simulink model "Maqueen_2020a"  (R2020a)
settings: Solver=VariableStepAuto  StartTime=0.0  StopTime=2  RelTol=1e-3
model workspace: external: MAT-File (data not in the file)
undefined symbols (not defined in the file or in its folder): deg, kg, m, mm, N, rad, s, smiData, X, Y, Z
libraries: sm_lib x459, fl_lib x12, nesl_utility x10
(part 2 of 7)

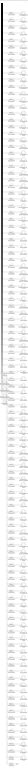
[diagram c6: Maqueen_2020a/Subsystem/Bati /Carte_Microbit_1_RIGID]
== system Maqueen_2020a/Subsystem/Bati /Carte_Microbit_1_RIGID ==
  Antenne_1_RIGID : Subsystem
  Assembly2_1_RIGID : Subsystem
  Button_assembly_microbit_1_RIGID : Subsystem
  Button_assembly_microbit_2_RIGID : Subsystem
  Button_assembly_microbit_3_RIGID : Subsystem
  Carte_microbit_1_RIGID : Subsystem
  Circuit_integre_1_1_RIGID : Subsystem
  Circuit_integre_2_1_RIGID : Subsystem
  Circuit_integre_3_1_RIGID : Subsystem
  Circuit_integre_3_2_RIGID : Subsystem
  Circuit_integre_4_1_RIGID : Subsystem
  Circuit_integre_4_2_RIGID : Subsystem
  Circuit_integre_5_1_RIGID : Subsystem
  Condensateur_1_RIGID : Subsystem
  Condensateur_2_RIGID : Subsystem
  Condensateur_3_RIGID : Subsystem
  Condensateur_4_RIGID : Subsystem
  Condensateur_5_RIGID : Subsystem
  Condensateur_6_RIGID : Subsystem
  Condensateur_cylindrique_10_RIGID : Subsystem
  Condensateur_cylindrique_11_RIGID : Subsystem
  Condensateur_cylindrique_12_RIGID : Subsystem
  Condensateur_cylindrique_13_RIGID : Subsystem
  Condensateur_cylindrique_14_RIGID : Subsystem
  Condensateur_cylindrique_15_RIGID : Subsystem
  Condensateur_cylindrique_16_RIGID : Subsystem
  Condensateur_cylindrique_17_RIGID : Subsystem
  Condensateur_cylindrique_18_RIGID : Subsystem
  Condensateur_cylindrique_19_RIGID : Subsystem
  Condensateur_cylindrique_1_RIGID : Subsystem
  Condensateur_cylindrique_20_RIGID : Subsystem
  Condensateur_cylindrique_2_RIGID : Subsystem
  Condensateur_cylindrique_3_RIGID : Subsystem
  Condensateur_cylindrique_4_RIGID : Subsystem
  Condensateur_cylindrique_5_RIGID : Subsystem
  Condensateur_cylindrique_6_RIGID : Subsystem
  Condensateur_cylindrique_7_RIGID : Subsystem
  Condensateur_cylindrique_8_RIGID : Subsystem
  Condensateur_cylindrique_9_RIGID : Subsystem
  Connecteur_alimentation_1_RIGID : Subsystem
  LED_10_RIGID : Subsystem
  LED_11_RIGID : Subsystem
  LED_12_RIGID : Subsystem
  LED_13_RIGID : Subsystem
  LED_14_RIGID : Subsystem
  LED_15_RIGID : Subsystem
  LED_16_RIGID : Subsystem
  LED_17_RIGID : Subsystem
  LED_18_RIGID : Subsystem
  LED_19_RIGID : Subsystem
  LED_1_RIGID : Subsystem
  LED_20_RIGID : Subsystem
  LED_21_RIGID : Subsystem
  LED_22_RIGID : Subsystem
  LED_23_RIGID : Subsystem
  LED_24_RIGID : Subsystem
  LED_25_RIGID : Subsystem
  LED_2_RIGID : Subsystem
  LED_3_RIGID : Subsystem
  LED_4_RIGID : Subsystem
  LED_5_RIGID : Subsystem
  LED_6_RIGID : Subsystem
  LED_7_RIGID : Subsystem
  LED_8_RIGID : Subsystem
  LED_9_RIGID : Subsystem
  Lignes_face_arrire_1_RIGID : Subsystem
  Pins_1_RIGID : Subsystem
  Pins_2_RIGID : Subsystem
  ReferenceFrame : sm_lib/Frames and Transforms/Reference Frame
  Resistance_10_RIGID : Subsystem
  Resistance_11_RIGID : Subsystem
  Resistance_12_RIGID : Subsystem
  Resistance_13_RIGID : Subsystem
  Resistance_14_RIGID : Subsystem
  Resistance_15_RIGID : Subsystem
  Resistance_16_RIGID : Subsystem
  Resistance_17_RIGID : Subsystem
  Resistance_18_RIGID : Subsystem
  Resistance_19_RIGID : Subsystem
  Resistance_1_RIGID : Subsystem
  Resistance_20_RIGID : Subsystem
  Resistance_21_RIGID : Subsystem
  Resistance_22_RIGID : Subsystem
  Resistance_23_RIGID : Subsystem
  Resistance_24_RIGID : Subsystem
  Resistance_25_RIGID : Subsystem
  Resistance_26_RIGID : Subsystem
  Resistance_27_RIGID : Subsystem
  Resistance_28_RIGID : Subsystem
  Resistance_29_RIGID : Subsystem
  Resistance_2_RIGID : Subsystem
  Resistance_30_RIGID : Subsystem
  Resistance_31_RIGID : Subsystem
  Resistance_32_RIGID : Subsystem
  Resistance_33_RIGID : Subsystem
  Resistance_34_RIGID : Subsystem
  Resistance_35_RIGID : Subsystem
  Resistance_36_RIGID : Subsystem
  Resistance_37_RIGID : Subsystem
  Resistance_38_RIGID : Subsystem
  Resistance_39_RIGID : Subsystem
  Resistance_3_RIGID : Subsystem
  Resistance_40_RIGID : Subsystem
  Resistance_41_RIGID : Subsystem
  Resistance_42_RIGID : Subsystem
  Resistance_43_RIGID : Subsystem
  Resistance_44_RIGID : Subsystem
  Resistance_45_RIGID : Subsystem
  Resistance_4_RIGID : Subsystem
  Resistance_5_RIGID : Subsystem
  Resistance_6_RIGID : Subsystem
  Resistance_7_RIGID : Subsystem
  Resistance_8_RIGID : Subsystem
  Resistance_9_RIGID : Subsystem
  Slot_condensateur_1_RIGID : Subsystem
  Texte_derriere_1_RIGID : Subsystem
  Texte_face_devant_1_RIGID : Subsystem
  Transform : sm_lib/Frames and Transforms/Rigid Transform  TranslationMethod=Cartesian  TranslationStandardOffset=0  TranslationLengthUnit=mm  TranslationStandardAxis=+Z  TranslationCartesianOffset=smiData.RigidTransform(6).translation  TranslationROffset=0  TranslationROffsetUnits=m  TranslationZOffset=0  TranslationZOffsetUnits=m  TranslationThetaOffset=0  TranslationThetaOffsetUnits=deg  RotationMethod=ArbitraryAxis  RotationAngleUnits=rad  RotationStandardAxis=+Z  RotationAngle=smiData.RigidTransform(6).angle  RotationArbitraryAxis=smiData.RigidTransform(6).axis  FollAlignAxisA=+X  BaseAlignAxisA=+Y  FollAlignAxisB=+Y  BaseAlignAxisB=+Z  RotationSequenceAxes=FollowerAxes  RotationSequence=XYX  RotationSequenceAngles=[0 0 0]  RotationSequenceAnglesUnits=deg  RotationMatrix=[1 0 0; 0 1 0; 0 0 1]
  Transform1 : sm_lib/Frames and Transforms/Rigid Transform  TranslationMethod=Cartesian  TranslationStandardOffset=0  TranslationLengthUnit=mm  TranslationStandardAxis=+Z  TranslationCartesianOffset=smiData.RigidTransform(29).translation  TranslationROffset=0  TranslationROffsetUnits=m  TranslationZOffset=0  TranslationZOffsetUnits=m  TranslationThetaOffset=0  TranslationThetaOffsetUnits=deg  RotationMethod=ArbitraryAxis  RotationAngleUnits=rad  RotationStandardAxis=+Z  RotationAngle=smiData.RigidTransform(29).angle  RotationArbitraryAxis=smiData.RigidTransform(29).axis  FollAlignAxisA=+X  BaseAlignAxisA=+Y  FollAlignAxisB=+Y  BaseAlignAxisB=+Z  RotationSequenceAxes=FollowerAxes  RotationSequence=XYX  RotationSequenceAngles=[0 0 0]  RotationSequenceAnglesUnits=deg  RotationMatrix=[1 0 0; 0 1 0; 0 0 1]
  Transform10 : sm_lib/Frames and Transforms/Rigid Transform  TranslationMethod=Cartesian  TranslationStandardOffset=0  TranslationLengthUnit=mm  TranslationStandardAxis=+Z  TranslationCartesianOffset=smiData.RigidTransform(38).translation  TranslationROffset=0  TranslationROffsetUnits=m  TranslationZOffset=0  TranslationZOffsetUnits=m  TranslationThetaOffset=0  TranslationThetaOffsetUnits=deg  RotationMethod=ArbitraryAxis  RotationAngleUnits=rad  RotationStandardAxis=+Z  RotationAngle=smiData.RigidTransform(38).angle  RotationArbitraryAxis=smiData.RigidTransform(38).axis  FollAlignAxisA=+X  BaseAlignAxisA=+Y  FollAlignAxisB=+Y  BaseAlignAxisB=+Z  RotationSequenceAxes=FollowerAxes  RotationSequence=XYX  RotationSequenceAngles=[0 0 0]  RotationSequenceAnglesUnits=deg  RotationMatrix=[1 0 0; 0 1 0; 0 0 1]
  Transform100 : sm_lib/Frames and Transforms/Rigid Transform  TranslationMethod=Cartesian  TranslationStandardOffset=0  TranslationLengthUnit=mm  TranslationStandardAxis=+Z  TranslationCartesianOffset=smiData.RigidTransform(137).translation  TranslationROffset=0  TranslationROffsetUnits=m  TranslationZOffset=0  TranslationZOffsetUnits=m  TranslationThetaOffset=0  TranslationThetaOffsetUnits=deg  RotationMethod=ArbitraryAxis  RotationAngleUnits=rad  RotationStandardAxis=+Z  RotationAngle=smiData.RigidTransform(137).angle  RotationArbitraryAxis=smiData.RigidTransform(137).axis  FollAlignAxisA=+X  BaseAlignAxisA=+Y  FollAlignAxisB=+Y  BaseAlignAxisB=+Z  RotationSequenceAxes=FollowerAxes  RotationSequence=XYX  RotationSequenceAngles=[0 0 0]  RotationSequenceAnglesUnits=deg  RotationMatrix=[1 0 0; 0 1 0; 0 0 1]
  Transform101 : sm_lib/Frames and Transforms/Rigid Transform  TranslationMethod=Cartesian  TranslationStandardOffset=0  TranslationLengthUnit=mm  TranslationStandardAxis=+Z  TranslationCartesianOffset=smiData.RigidTransform(138).translation  TranslationROffset=0  TranslationROffsetUnits=m  TranslationZOffset=0  TranslationZOffsetUnits=m  TranslationThetaOffset=0  TranslationThetaOffsetUnits=deg  RotationMethod=ArbitraryAxis  RotationAngleUnits=rad  RotationStandardAxis=+Z  RotationAngle=smiData.RigidTransform(138).angle  RotationArbitraryAxis=smiData.RigidTransform(138).axis  FollAlignAxisA=+X  BaseAlignAxisA=+Y  FollAlignAxisB=+Y  BaseAlignAxisB=+Z  RotationSequenceAxes=FollowerAxes  RotationSequence=XYX  RotationSequenceAngles=[0 0 0]  RotationSequenceAnglesUnits=deg  RotationMatrix=[1 0 0; 0 1 0; 0 0 1]
  Transform102 : sm_lib/Frames and Transforms/Rigid Transform  TranslationMethod=Cartesian  TranslationStandardOffset=0  TranslationLengthUnit=mm  TranslationStandardAxis=+Z  TranslationCartesianOffset=smiData.RigidTransform(139).translation  TranslationROffset=0  TranslationROffsetUnits=m  TranslationZOffset=0  TranslationZOffsetUnits=m  TranslationThetaOffset=0  TranslationThetaOffsetUnits=deg  RotationMethod=ArbitraryAxis  RotationAngleUnits=rad  RotationStandardAxis=+Z  RotationAngle=smiData.RigidTransform(139).angle  RotationArbitraryAxis=smiData.RigidTransform(139).axis  FollAlignAxisA=+X  BaseAlignAxisA=+Y  FollAlignAxisB=+Y  BaseAlignAxisB=+Z  RotationSequenceAxes=FollowerAxes  RotationSequence=XYX  RotationSequenceAngles=[0 0 0]  RotationSequenceAnglesUnits=deg  RotationMatrix=[1 0 0; 0 1 0; 0 0 1]
  Transform103 : sm_lib/Frames and Transforms/Rigid Transform  TranslationMethod=Cartesian  TranslationStandardOffset=0  TranslationLengthUnit=mm  TranslationStandardAxis=+Z  TranslationCartesianOffset=smiData.RigidTransform(140).translation  TranslationROffset=0  TranslationROffsetUnits=m  TranslationZOffset=0  TranslationZOffsetUnits=m  TranslationThetaOffset=0  TranslationThetaOffsetUnits=deg  RotationMethod=ArbitraryAxis  RotationAngleUnits=rad  RotationStandardAxis=+Z  RotationAngle=smiData.RigidTransform(140).angle  RotationArbitraryAxis=smiData.RigidTransform(140).axis  FollAlignAxisA=+X  BaseAlignAxisA=+Y  FollAlignAxisB=+Y  BaseAlignAxisB=+Z  RotationSequenceAxes=FollowerAxes  RotationSequence=XYX  RotationSequenceAngles=[0 0 0]  RotationSequenceAnglesUnits=deg  RotationMatrix=[1 0 0; 0 1 0; 0 0 1]
  Transform104 : sm_lib/Frames and Transforms/Rigid Transform  TranslationMethod=Cartesian  TranslationStandardOffset=0  TranslationLengthUnit=mm  TranslationStandardAxis=+Z  TranslationCartesianOffset=smiData.RigidTransform(145).translation  TranslationROffset=0  TranslationROffsetUnits=m  TranslationZOffset=0  TranslationZOffsetUnits=m  TranslationThetaOffset=0  TranslationThetaOffsetUnits=deg  RotationMethod=ArbitraryAxis  RotationAngleUnits=rad  RotationStandardAxis=+Z  RotationAngle=smiData.RigidTransform(145).angle  RotationArbitraryAxis=smiData.RigidTransform(145).axis  FollAlignAxisA=+X  BaseAlignAxisA=+Y  FollAlignAxisB=+Y  BaseAlignAxisB=+Z  RotationSequenceAxes=FollowerAxes  RotationSequence=XYX  RotationSequenceAngles=[0 0 0]  RotationSequenceAnglesUnits=deg  RotationMatrix=[1 0 0; 0 1 0; 0 0 1]
  Transform105 : sm_lib/Frames and Transforms/Rigid Transform  TranslationMethod=Cartesian  TranslationStandardOffset=0  TranslationLengthUnit=mm  TranslationStandardAxis=+Z  TranslationCartesianOffset=smiData.RigidTransform(150).translation  TranslationROffset=0  TranslationROffsetUnits=m  TranslationZOffset=0  TranslationZOffsetUnits=m  TranslationThetaOffset=0  TranslationThetaOffsetUnits=deg  RotationMethod=ArbitraryAxis  RotationAngleUnits=rad  RotationStandardAxis=+Z  RotationAngle=smiData.RigidTransform(150).angle  RotationArbitraryAxis=smiData.RigidTransform(150).axis  FollAlignAxisA=+X  BaseAlignAxisA=+Y  FollAlignAxisB=+Y  BaseAlignAxisB=+Z  RotationSequenceAxes=FollowerAxes  RotationSequence=XYX  RotationSequenceAngles=[0 0 0]  RotationSequenceAnglesUnits=deg  RotationMatrix=[1 0 0; 0 1 0; 0 0 1]
  Transform106 : sm_lib/Frames and Transforms/Rigid Transform  TranslationMethod=Cartesian  TranslationStandardOffset=0  TranslationLengthUnit=mm  TranslationStandardAxis=+Z  TranslationCartesianOffset=smiData.RigidTransform(151).translation  TranslationROffset=0  TranslationROffsetUnits=m  TranslationZOffset=0  TranslationZOffsetUnits=m  TranslationThetaOffset=0  TranslationThetaOffsetUnits=deg  RotationMethod=ArbitraryAxis  RotationAngleUnits=rad  RotationStandardAxis=+Z  RotationAngle=smiData.RigidTransform(151).angle  RotationArbitraryAxis=smiData.RigidTransform(151).axis  FollAlignAxisA=+X  BaseAlignAxisA=+Y  FollAlignAxisB=+Y  BaseAlignAxisB=+Z  RotationSequenceAxes=FollowerAxes  RotationSequence=XYX  RotationSequenceAngles=[0 0 0]  RotationSequenceAnglesUnits=deg  RotationMatrix=[1 0 0; 0 1 0; 0 0 1]
  Transform107 : sm_lib/Frames and Transforms/Rigid Transform  TranslationMethod=Cartesian  TranslationStandardOffset=0  TranslationLengthUnit=mm  TranslationStandardAxis=+Z  TranslationCartesianOffset=smiData.RigidTransform(152).translation  TranslationROffset=0  TranslationROffsetUnits=m  TranslationZOffset=0  TranslationZOffsetUnits=m  TranslationThetaOffset=0  TranslationThetaOffsetUnits=deg  RotationMethod=ArbitraryAxis  RotationAngleUnits=rad  RotationStandardAxis=+Z  RotationAngle=smiData.RigidTransform(152).angle  RotationArbitraryAxis=smiData.RigidTransform(152).axis  FollAlignAxisA=+X  BaseAlignAxisA=+Y  FollAlignAxisB=+Y  BaseAlignAxisB=+Z  RotationSequenceAxes=FollowerAxes  RotationSequence=XYX  RotationSequenceAngles=[0 0 0]  RotationSequenceAnglesUnits=deg  RotationMatrix=[1 0 0; 0 1 0; 0 0 1]
  Transform108 : sm_lib/Frames and Transforms/Rigid Transform  TranslationMethod=Cartesian  TranslationStandardOffset=0  TranslationLengthUnit=mm  TranslationStandardAxis=+Z  TranslationCartesianOffset=smiData.RigidTransform(153).translation  TranslationROffset=0  TranslationROffsetUnits=m  TranslationZOffset=0  TranslationZOffsetUnits=m  TranslationThetaOffset=0  TranslationThetaOffsetUnits=deg  RotationMethod=ArbitraryAxis  RotationAngleUnits=rad  RotationStandardAxis=+Z  RotationAngle=smiData.RigidTransform(153).angle  RotationArbitraryAxis=smiData.RigidTransform(153).axis  FollAlignAxisA=+X  BaseAlignAxisA=+Y  FollAlignAxisB=+Y  BaseAlignAxisB=+Z  RotationSequenceAxes=FollowerAxes  RotationSequence=XYX  RotationSequenceAngles=[0 0 0]  RotationSequenceAnglesUnits=deg  RotationMatrix=[1 0 0; 0 1 0; 0 0 1]
  Transform109 : sm_lib/Frames and Transforms/Rigid Transform  TranslationMethod=Cartesian  TranslationStandardOffset=0  TranslationLengthUnit=mm  TranslationStandardAxis=+Z  TranslationCartesianOffset=smiData.RigidTransform(154).translation  TranslationROffset=0  TranslationROffsetUnits=m  TranslationZOffset=0  TranslationZOffsetUnits=m  TranslationThetaOffset=0  TranslationThetaOffsetUnits=deg  RotationMethod=ArbitraryAxis  RotationAngleUnits=rad  RotationStandardAxis=+Z  RotationAngle=smiData.RigidTransform(154).angle  RotationArbitraryAxis=smiData.RigidTransform(154).axis  FollAlignAxisA=+X  BaseAlignAxisA=+Y  FollAlignAxisB=+Y  BaseAlignAxisB=+Z  RotationSequenceAxes=FollowerAxes  RotationSequence=XYX  RotationSequenceAngles=[0 0 0]  RotationSequenceAnglesUnits=deg  RotationMatrix=[1 0 0; 0 1 0; 0 0 1]
  Transform11 : sm_lib/Frames and Transforms/Rigid Transform  TranslationMethod=Cartesian  TranslationStandardOffset=0  TranslationLengthUnit=mm  TranslationStandardAxis=+Z  TranslationCartesianOffset=smiData.RigidTransform(39).translation  TranslationROffset=0  TranslationROffsetUnits=m  TranslationZOffset=0  TranslationZOffsetUnits=m  TranslationThetaOffset=0  TranslationThetaOffsetUnits=deg  RotationMethod=ArbitraryAxis  RotationAngleUnits=rad  RotationStandardAxis=+Z  RotationAngle=smiData.RigidTransform(39).angle  RotationArbitraryAxis=smiData.RigidTransform(39).axis  FollAlignAxisA=+X  BaseAlignAxisA=+Y  FollAlignAxisB=+Y  BaseAlignAxisB=+Z  RotationSequenceAxes=FollowerAxes  RotationSequence=XYX  RotationSequenceAngles=[0 0 0]  RotationSequenceAnglesUnits=deg  RotationMatrix=[1 0 0; 0 1 0; 0 0 1]
  Transform110 : sm_lib/Frames and Transforms/Rigid Transform  TranslationMethod=Cartesian  TranslationStandardOffset=0  TranslationLengthUnit=mm  TranslationStandardAxis=+Z  TranslationCartesianOffset=smiData.RigidTransform(155).translation  TranslationROffset=0  TranslationROffsetUnits=m  TranslationZOffset=0  TranslationZOffsetUnits=m  TranslationThetaOffset=0  TranslationThetaOffsetUnits=deg  RotationMethod=ArbitraryAxis  RotationAngleUnits=rad  RotationStandardAxis=+Z  RotationAngle=smiData.RigidTransform(155).angle  RotationArbitraryAxis=smiData.RigidTransform(155).axis  FollAlignAxisA=+X  BaseAlignAxisA=+Y  FollAlignAxisB=+Y  BaseAlignAxisB=+Z  RotationSequenceAxes=FollowerAxes  RotationSequence=XYX  RotationSequenceAngles=[0 0 0]  RotationSequenceAnglesUnits=deg  RotationMatrix=[1 0 0; 0 1 0; 0 0 1]
  Transform111 : sm_lib/Frames and Transforms/Rigid Transform  TranslationMethod=Cartesian  TranslationStandardOffset=0  TranslationLengthUnit=mm  TranslationStandardAxis=+Z  TranslationCartesianOffset=smiData.RigidTransform(156).translation  TranslationROffset=0  TranslationROffsetUnits=m  TranslationZOffset=0  TranslationZOffsetUnits=m  TranslationThetaOffset=0  TranslationThetaOffsetUnits=deg  RotationMethod=ArbitraryAxis  RotationAngleUnits=rad  RotationStandardAxis=+Z  RotationAngle=smiData.RigidTransform(156).angle  RotationArbitraryAxis=smiData.RigidTransform(156).axis  FollAlignAxisA=+X  BaseAlignAxisA=+Y  FollAlignAxisB=+Y  BaseAlignAxisB=+Z  RotationSequenceAxes=FollowerAxes  RotationSequence=XYX  RotationSequenceAngles=[0 0 0]  RotationSequenceAnglesUnits=deg  RotationMatrix=[1 0 0; 0 1 0; 0 0 1]
  Transform112 : sm_lib/Frames and Transforms/Rigid Transform  TranslationMethod=Cartesian  TranslationStandardOffset=0  TranslationLengthUnit=mm  TranslationStandardAxis=+Z  TranslationCartesianOffset=smiData.RigidTransform(157).translation  TranslationROffset=0  TranslationROffsetUnits=m  TranslationZOffset=0  TranslationZOffsetUnits=m  TranslationThetaOffset=0  TranslationThetaOffsetUnits=deg  RotationMethod=ArbitraryAxis  RotationAngleUnits=rad  RotationStandardAxis=+Z  RotationAngle=smiData.RigidTransform(157).angle  RotationArbitraryAxis=smiData.RigidTransform(157).axis  FollAlignAxisA=+X  BaseAlignAxisA=+Y  FollAlignAxisB=+Y  BaseAlignAxisB=+Z  RotationSequenceAxes=FollowerAxes  RotationSequence=XYX  RotationSequenceAngles=[0 0 0]  RotationSequenceAnglesUnits=deg  RotationMatrix=[1 0 0; 0 1 0; 0 0 1]
  Transform113 : sm_lib/Frames and Transforms/Rigid Transform  TranslationMethod=Cartesian  TranslationStandardOffset=0  TranslationLengthUnit=mm  TranslationStandardAxis=+Z  TranslationCartesianOffset=smiData.RigidTransform(158).translation  TranslationROffset=0  TranslationROffsetUnits=m  TranslationZOffset=0  TranslationZOffsetUnits=m  TranslationThetaOffset=0  TranslationThetaOffsetUnits=deg  RotationMethod=ArbitraryAxis  RotationAngleUnits=rad  RotationStandardAxis=+Z  RotationAngle=smiData.RigidTransform(158).angle  RotationArbitraryAxis=smiData.RigidTransform(158).axis  FollAlignAxisA=+X  BaseAlignAxisA=+Y  FollAlignAxisB=+Y  BaseAlignAxisB=+Z  RotationSequenceAxes=FollowerAxes  RotationSequence=XYX  RotationSequenceAngles=[0 0 0]  RotationSequenceAnglesUnits=deg  RotationMatrix=[1 0 0; 0 1 0; 0 0 1]
  Transform12 : sm_lib/Frames and Transforms/Rigid Transform  TranslationMethod=Cartesian  TranslationStandardOffset=0  TranslationLengthUnit=mm  TranslationStandardAxis=+Z  TranslationCartesianOffset=smiData.RigidTransform(40).translation  TranslationROffset=0  TranslationROffsetUnits=m  TranslationZOffset=0  TranslationZOffsetUnits=m  TranslationThetaOffset=0  TranslationThetaOffsetUnits=deg  RotationMethod=ArbitraryAxis  RotationAngleUnits=rad  RotationStandardAxis=+Z  RotationAngle=smiData.RigidTransform(40).angle  RotationArbitraryAxis=smiData.RigidTransform(40).axis  FollAlignAxisA=+X  BaseAlignAxisA=+Y  FollAlignAxisB=+Y  BaseAlignAxisB=+Z  RotationSequenceAxes=FollowerAxes  RotationSequence=XYX  RotationSequenceAngles=[0 0 0]  RotationSequenceAnglesUnits=deg  RotationMatrix=[1 0 0; 0 1 0; 0 0 1]
  Transform13 : sm_lib/Frames and Transforms/Rigid Transform  TranslationMethod=Cartesian  TranslationStandardOffset=0  TranslationLengthUnit=mm  TranslationStandardAxis=+Z  TranslationCartesianOffset=smiData.RigidTransform(41).translation  TranslationROffset=0  TranslationROffsetUnits=m  TranslationZOffset=0  TranslationZOffsetUnits=m  TranslationThetaOffset=0  TranslationThetaOffsetUnits=deg  RotationMethod=ArbitraryAxis  RotationAngleUnits=rad  RotationStandardAxis=+Z  RotationAngle=smiData.RigidTransform(41).angle  RotationArbitraryAxis=smiData.RigidTransform(41).axis  FollAlignAxisA=+X  BaseAlignAxisA=+Y  FollAlignAxisB=+Y  BaseAlignAxisB=+Z  RotationSequenceAxes=FollowerAxes  RotationSequence=XYX  RotationSequenceAngles=[0 0 0]  RotationSequenceAnglesUnits=deg  RotationMatrix=[1 0 0; 0 1 0; 0 0 1]
  Transform14 : sm_lib/Frames and Transforms/Rigid Transform  TranslationMethod=Cartesian  TranslationStandardOffset=0  TranslationLengthUnit=mm  TranslationStandardAxis=+Z  TranslationCartesianOffset=smiData.RigidTransform(42).translation  TranslationROffset=0  TranslationROffsetUnits=m  TranslationZOffset=0  TranslationZOffsetUnits=m  TranslationThetaOffset=0  TranslationThetaOffsetUnits=deg  RotationMethod=ArbitraryAxis  RotationAngleUnits=rad  RotationStandardAxis=+Z  RotationAngle=smiData.RigidTransform(42).angle  RotationArbitraryAxis=smiData.RigidTransform(42).axis  FollAlignAxisA=+X  BaseAlignAxisA=+Y  FollAlignAxisB=+Y  BaseAlignAxisB=+Z  RotationSequenceAxes=FollowerAxes  RotationSequence=XYX  RotationSequenceAngles=[0 0 0]  RotationSequenceAnglesUnits=deg  RotationMatrix=[1 0 0; 0 1 0; 0 0 1]
  Transform15 : sm_lib/Frames and Transforms/Rigid Transform  TranslationMethod=Cartesian  TranslationStandardOffset=0  TranslationLengthUnit=mm  TranslationStandardAxis=+Z  TranslationCartesianOffset=smiData.RigidTransform(43).translation  TranslationROffset=0  TranslationROffsetUnits=m  TranslationZOffset=0  TranslationZOffsetUnits=m  TranslationThetaOffset=0  TranslationThetaOffsetUnits=deg  RotationMethod=ArbitraryAxis  RotationAngleUnits=rad  RotationStandardAxis=+Z  RotationAngle=smiData.RigidTransform(43).angle  RotationArbitraryAxis=smiData.RigidTransform(43).axis  FollAlignAxisA=+X  BaseAlignAxisA=+Y  FollAlignAxisB=+Y  BaseAlignAxisB=+Z  RotationSequenceAxes=FollowerAxes  RotationSequence=XYX  RotationSequenceAngles=[0 0 0]  RotationSequenceAnglesUnits=deg  RotationMatrix=[1 0 0; 0 1 0; 0 0 1]
  Transform16 : sm_lib/Frames and Transforms/Rigid Transform  TranslationMethod=Cartesian  TranslationStandardOffset=0  TranslationLengthUnit=mm  TranslationStandardAxis=+Z  TranslationCartesianOffset=smiData.RigidTransform(44).translation  TranslationROffset=0  TranslationROffsetUnits=m  TranslationZOffset=0  TranslationZOffsetUnits=m  TranslationThetaOffset=0  TranslationThetaOffsetUnits=deg  RotationMethod=ArbitraryAxis  RotationAngleUnits=rad  RotationStandardAxis=+Z  RotationAngle=smiData.RigidTransform(44).angle  RotationArbitraryAxis=smiData.RigidTransform(44).axis  FollAlignAxisA=+X  BaseAlignAxisA=+Y  FollAlignAxisB=+Y  BaseAlignAxisB=+Z  RotationSequenceAxes=FollowerAxes  RotationSequence=XYX  RotationSequenceAngles=[0 0 0]  RotationSequenceAnglesUnits=deg  RotationMatrix=[1 0 0; 0 1 0; 0 0 1]
  Transform17 : sm_lib/Frames and Transforms/Rigid Transform  TranslationMethod=Cartesian  TranslationStandardOffset=0  TranslationLengthUnit=mm  TranslationStandardAxis=+Z  TranslationCartesianOffset=smiData.RigidTransform(45).translation  TranslationROffset=0  TranslationROffsetUnits=m  TranslationZOffset=0  TranslationZOffsetUnits=m  TranslationThetaOffset=0  TranslationThetaOffsetUnits=deg  RotationMethod=ArbitraryAxis  RotationAngleUnits=rad  RotationStandardAxis=+Z  RotationAngle=smiData.RigidTransform(45).angle  RotationArbitraryAxis=smiData.RigidTransform(45).axis  FollAlignAxisA=+X  BaseAlignAxisA=+Y  FollAlignAxisB=+Y  BaseAlignAxisB=+Z  RotationSequenceAxes=FollowerAxes  RotationSequence=XYX  RotationSequenceAngles=[0 0 0]  RotationSequenceAnglesUnits=deg  RotationMatrix=[1 0 0; 0 1 0; 0 0 1]
  Transform18 : sm_lib/Frames and Transforms/Rigid Transform  TranslationMethod=Cartesian  TranslationStandardOffset=0  TranslationLengthUnit=mm  TranslationStandardAxis=+Z  TranslationCartesianOffset=smiData.RigidTransform(46).translation  TranslationROffset=0  TranslationROffsetUnits=m  TranslationZOffset=0  TranslationZOffsetUnits=m  TranslationThetaOffset=0  TranslationThetaOffsetUnits=deg  RotationMethod=ArbitraryAxis  RotationAngleUnits=rad  RotationStandardAxis=+Z  RotationAngle=smiData.RigidTransform(46).angle  RotationArbitraryAxis=smiData.RigidTransform(46).axis  FollAlignAxisA=+X  BaseAlignAxisA=+Y  FollAlignAxisB=+Y  BaseAlignAxisB=+Z  RotationSequenceAxes=FollowerAxes  RotationSequence=XYX  RotationSequenceAngles=[0 0 0]  RotationSequenceAnglesUnits=deg  RotationMatrix=[1 0 0; 0 1 0; 0 0 1]
  Transform19 : sm_lib/Frames and Transforms/Rigid Transform  TranslationMethod=Cartesian  TranslationStandardOffset=0  TranslationLengthUnit=mm  TranslationStandardAxis=+Z  TranslationCartesianOffset=smiData.RigidTransform(47).translation  TranslationROffset=0  TranslationROffsetUnits=m  TranslationZOffset=0  TranslationZOffsetUnits=m  TranslationThetaOffset=0  TranslationThetaOffsetUnits=deg  RotationMethod=ArbitraryAxis  RotationAngleUnits=rad  RotationStandardAxis=+Z  RotationAngle=smiData.RigidTransform(47).angle  RotationArbitraryAxis=smiData.RigidTransform(47).axis  FollAlignAxisA=+X  BaseAlignAxisA=+Y  FollAlignAxisB=+Y  BaseAlignAxisB=+Z  RotationSequenceAxes=FollowerAxes  RotationSequence=XYX  RotationSequenceAngles=[0 0 0]  RotationSequenceAnglesUnits=deg  RotationMatrix=[1 0 0; 0 1 0; 0 0 1]
  Transform2 : sm_lib/Frames and Transforms/Rigid Transform  TranslationMethod=Cartesian  TranslationStandardOffset=0  TranslationLengthUnit=mm  TranslationStandardAxis=+Z  TranslationCartesianOffset=smiData.RigidTransform(30).translation  TranslationROffset=0  TranslationROffsetUnits=m  TranslationZOffset=0  TranslationZOffsetUnits=m  TranslationThetaOffset=0  TranslationThetaOffsetUnits=deg  RotationMethod=ArbitraryAxis  RotationAngleUnits=rad  RotationStandardAxis=+Z  RotationAngle=smiData.RigidTransform(30).angle  RotationArbitraryAxis=smiData.RigidTransform(30).axis  FollAlignAxisA=+X  BaseAlignAxisA=+Y  FollAlignAxisB=+Y  BaseAlignAxisB=+Z  RotationSequenceAxes=FollowerAxes  RotationSequence=XYX  RotationSequenceAngles=[0 0 0]  RotationSequenceAnglesUnits=deg  RotationMatrix=[1 0 0; 0 1 0; 0 0 1]
  Transform20 : sm_lib/Frames and Transforms/Rigid Transform  TranslationMethod=Cartesian  TranslationStandardOffset=0  TranslationLengthUnit=mm  TranslationStandardAxis=+Z  TranslationCartesianOffset=smiData.RigidTransform(48).translation  TranslationROffset=0  TranslationROffsetUnits=m  TranslationZOffset=0  TranslationZOffsetUnits=m  TranslationThetaOffset=0  TranslationThetaOffsetUnits=deg  RotationMethod=ArbitraryAxis  RotationAngleUnits=rad  RotationStandardAxis=+Z  RotationAngle=smiData.RigidTransform(48).angle  RotationArbitraryAxis=smiData.RigidTransform(48).axis  FollAlignAxisA=+X  BaseAlignAxisA=+Y  FollAlignAxisB=+Y  BaseAlignAxisB=+Z  RotationSequenceAxes=FollowerAxes  RotationSequence=XYX  RotationSequenceAngles=[0 0 0]  RotationSequenceAnglesUnits=deg  RotationMatrix=[1 0 0; 0 1 0; 0 0 1]
  Transform21 : sm_lib/Frames and Transforms/Rigid Transform  TranslationMethod=Cartesian  TranslationStandardOffset=0  TranslationLengthUnit=mm  TranslationStandardAxis=+Z  TranslationCartesianOffset=smiData.RigidTransform(49).translation  TranslationROffset=0  TranslationROffsetUnits=m  TranslationZOffset=0  TranslationZOffsetUnits=m  TranslationThetaOffset=0  TranslationThetaOffsetUnits=deg  RotationMethod=ArbitraryAxis  RotationAngleUnits=rad  RotationStandardAxis=+Z  RotationAngle=smiData.RigidTransform(49).angle  RotationArbitraryAxis=smiData.RigidTransform(49).axis  FollAlignAxisA=+X  BaseAlignAxisA=+Y  FollAlignAxisB=+Y  BaseAlignAxisB=+Z  RotationSequenceAxes=FollowerAxes  RotationSequence=XYX  RotationSequenceAngles=[0 0 0]  RotationSequenceAnglesUnits=deg  RotationMatrix=[1 0 0; 0 1 0; 0 0 1]
  Transform22 : sm_lib/Frames and Transforms/Rigid Transform  TranslationMethod=Cartesian  TranslationStandardOffset=0  TranslationLengthUnit=mm  TranslationStandardAxis=+Z  TranslationCartesianOffset=smiData.RigidTransform(50).translation  TranslationROffset=0  TranslationROffsetUnits=m  TranslationZOffset=0  TranslationZOffsetUnits=m  TranslationThetaOffset=0  TranslationThetaOffsetUnits=deg  RotationMethod=ArbitraryAxis  RotationAngleUnits=rad  RotationStandardAxis=+Z  RotationAngle=smiData.RigidTransform(50).angle  RotationArbitraryAxis=smiData.RigidTransform(50).axis  FollAlignAxisA=+X  BaseAlignAxisA=+Y  FollAlignAxisB=+Y  BaseAlignAxisB=+Z  RotationSequenceAxes=FollowerAxes  RotationSequence=XYX  RotationSequenceAngles=[0 0 0]  RotationSequenceAnglesUnits=deg  RotationMatrix=[1 0 0; 0 1 0; 0 0 1]
  Transform23 : sm_lib/Frames and Transforms/Rigid Transform  TranslationMethod=Cartesian  TranslationStandardOffset=0  TranslationLengthUnit=mm  TranslationStandardAxis=+Z  TranslationCartesianOffset=smiData.RigidTransform(51).translation  TranslationROffset=0  TranslationROffsetUnits=m  TranslationZOffset=0  TranslationZOffsetUnits=m  TranslationThetaOffset=0  TranslationThetaOffsetUnits=deg  RotationMethod=ArbitraryAxis  RotationAngleUnits=rad  RotationStandardAxis=+Z  RotationAngle=smiData.RigidTransform(51).angle  RotationArbitraryAxis=smiData.RigidTransform(51).axis  FollAlignAxisA=+X  BaseAlignAxisA=+Y  FollAlignAxisB=+Y  BaseAlignAxisB=+Z  RotationSequenceAxes=FollowerAxes  RotationSequence=XYX  RotationSequenceAngles=[0 0 0]  RotationSequenceAnglesUnits=deg  RotationMatrix=[1 0 0; 0 1 0; 0 0 1]
  Transform24 : sm_lib/Frames and Transforms/Rigid Transform  TranslationMethod=Cartesian  TranslationStandardOffset=0  TranslationLengthUnit=mm  TranslationStandardAxis=+Z  TranslationCartesianOffset=smiData.RigidTransform(52).translation  TranslationROffset=0  TranslationROffsetUnits=m  TranslationZOffset=0  TranslationZOffsetUnits=m  TranslationThetaOffset=0  TranslationThetaOffsetUnits=deg  RotationMethod=ArbitraryAxis  RotationAngleUnits=rad  RotationStandardAxis=+Z  RotationAngle=smiData.RigidTransform(52).angle  RotationArbitraryAxis=smiData.RigidTransform(52).axis  FollAlignAxisA=+X  BaseAlignAxisA=+Y  FollAlignAxisB=+Y  BaseAlignAxisB=+Z  RotationSequenceAxes=FollowerAxes  RotationSequence=XYX  RotationSequenceAngles=[0 0 0]  RotationSequenceAnglesUnits=deg  RotationMatrix=[1 0 0; 0 1 0; 0 0 1]
  Transform25 : sm_lib/Frames and Transforms/Rigid Transform  TranslationMethod=Cartesian  TranslationStandardOffset=0  TranslationLengthUnit=mm  TranslationStandardAxis=+Z  TranslationCartesianOffset=smiData.RigidTransform(53).translation  TranslationROffset=0  TranslationROffsetUnits=m  TranslationZOffset=0  TranslationZOffsetUnits=m  TranslationThetaOffset=0  TranslationThetaOffsetUnits=deg  RotationMethod=ArbitraryAxis  RotationAngleUnits=rad  RotationStandardAxis=+Z  RotationAngle=smiData.RigidTransform(53).angle  RotationArbitraryAxis=smiData.RigidTransform(53).axis  FollAlignAxisA=+X  BaseAlignAxisA=+Y  FollAlignAxisB=+Y  BaseAlignAxisB=+Z  RotationSequenceAxes=FollowerAxes  RotationSequence=XYX  RotationSequenceAngles=[0 0 0]  RotationSequenceAnglesUnits=deg  RotationMatrix=[1 0 0; 0 1 0; 0 0 1]
  Transform26 : sm_lib/Frames and Transforms/Rigid Transform  TranslationMethod=Cartesian  TranslationStandardOffset=0  TranslationLengthUnit=mm  TranslationStandardAxis=+Z  TranslationCartesianOffset=smiData.RigidTransform(54).translation  TranslationROffset=0  TranslationROffsetUnits=m  TranslationZOffset=0  TranslationZOffsetUnits=m  TranslationThetaOffset=0  TranslationThetaOffsetUnits=deg  RotationMethod=ArbitraryAxis  RotationAngleUnits=rad  RotationStandardAxis=+Z  RotationAngle=smiData.RigidTransform(54).angle  RotationArbitraryAxis=smiData.RigidTransform(54).axis  FollAlignAxisA=+X  BaseAlignAxisA=+Y  FollAlignAxisB=+Y  BaseAlignAxisB=+Z  RotationSequenceAxes=FollowerAxes  RotationSequence=XYX  RotationSequenceAngles=[0 0 0]  RotationSequenceAnglesUnits=deg  RotationMatrix=[1 0 0; 0 1 0; 0 0 1]
  Transform27 : sm_lib/Frames and Transforms/Rigid Transform  TranslationMethod=Cartesian  TranslationStandardOffset=0  TranslationLengthUnit=mm  TranslationStandardAxis=+Z  TranslationCartesianOffset=smiData.RigidTransform(55).translation  TranslationROffset=0  TranslationROffsetUnits=m  TranslationZOffset=0  TranslationZOffsetUnits=m  TranslationThetaOffset=0  TranslationThetaOffsetUnits=deg  RotationMethod=ArbitraryAxis  RotationAngleUnits=rad  RotationStandardAxis=+Z  RotationAngle=smiData.RigidTransform(55).angle  RotationArbitraryAxis=smiData.RigidTransform(55).axis  FollAlignAxisA=+X  BaseAlignAxisA=+Y  FollAlignAxisB=+Y  BaseAlignAxisB=+Z  RotationSequenceAxes=FollowerAxes  RotationSequence=XYX  RotationSequenceAngles=[0 0 0]  RotationSequenceAnglesUnits=deg  RotationMatrix=[1 0 0; 0 1 0; 0 0 1]
  Transform28 : sm_lib/Frames and Transforms/Rigid Transform  TranslationMethod=Cartesian  TranslationStandardOffset=0  TranslationLengthUnit=mm  TranslationStandardAxis=+Z  TranslationCartesianOffset=smiData.RigidTransform(56).translation  TranslationROffset=0  TranslationROffsetUnits=m  TranslationZOffset=0  TranslationZOffsetUnits=m  TranslationThetaOffset=0  TranslationThetaOffsetUnits=deg  RotationMethod=ArbitraryAxis  RotationAngleUnits=rad  RotationStandardAxis=+Z  RotationAngle=smiData.RigidTransform(56).angle  RotationArbitraryAxis=smiData.RigidTransform(56).axis  FollAlignAxisA=+X  BaseAlignAxisA=+Y  FollAlignAxisB=+Y  BaseAlignAxisB=+Z  RotationSequenceAxes=FollowerAxes  RotationSequence=XYX  RotationSequenceAngles=[0 0 0]  RotationSequenceAnglesUnits=deg  RotationMatrix=[1 0 0; 0 1 0; 0 0 1]
  Transform29 : sm_lib/Frames and Transforms/Rigid Transform  TranslationMethod=Cartesian  TranslationStandardOffset=0  TranslationLengthUnit=mm  TranslationStandardAxis=+Z  TranslationCartesianOffset=smiData.RigidTransform(57).translation  TranslationROffset=0  TranslationROffsetUnits=m  TranslationZOffset=0  TranslationZOffsetUnits=m  TranslationThetaOffset=0  TranslationThetaOffsetUnits=deg  RotationMethod=ArbitraryAxis  RotationAngleUnits=rad  RotationStandardAxis=+Z  RotationAngle=smiData.RigidTransform(57).angle  RotationArbitraryAxis=smiData.RigidTransform(57).axis  FollAlignAxisA=+X  BaseAlignAxisA=+Y  FollAlignAxisB=+Y  BaseAlignAxisB=+Z  RotationSequenceAxes=FollowerAxes  RotationSequence=XYX  RotationSequenceAngles=[0 0 0]  RotationSequenceAnglesUnits=deg  RotationMatrix=[1 0 0; 0 1 0; 0 0 1]
  Transform3 : sm_lib/Frames and Transforms/Rigid Transform  TranslationMethod=Cartesian  TranslationStandardOffset=0  TranslationLengthUnit=mm  TranslationStandardAxis=+Z  TranslationCartesianOffset=smiData.RigidTransform(31).translation  TranslationROffset=0  TranslationROffsetUnits=m  TranslationZOffset=0  TranslationZOffsetUnits=m  TranslationThetaOffset=0  TranslationThetaOffsetUnits=deg  RotationMethod=ArbitraryAxis  RotationAngleUnits=rad  RotationStandardAxis=+Z  RotationAngle=smiData.RigidTransform(31).angle  RotationArbitraryAxis=smiData.RigidTransform(31).axis  FollAlignAxisA=+X  BaseAlignAxisA=+Y  FollAlignAxisB=+Y  BaseAlignAxisB=+Z  RotationSequenceAxes=FollowerAxes  RotationSequence=XYX  RotationSequenceAngles=[0 0 0]  RotationSequenceAnglesUnits=deg  RotationMatrix=[1 0 0; 0 1 0; 0 0 1]
  Transform30 : sm_lib/Frames and Transforms/Rigid Transform  TranslationMethod=Cartesian  TranslationStandardOffset=0  TranslationLengthUnit=mm  TranslationStandardAxis=+Z  TranslationCartesianOffset=smiData.RigidTransform(58).translation  TranslationROffset=0  TranslationROffsetUnits=m  TranslationZOffset=0  TranslationZOffsetUnits=m  TranslationThetaOffset=0  TranslationThetaOffsetUnits=deg  RotationMethod=ArbitraryAxis  RotationAngleUnits=rad  RotationStandardAxis=+Z  RotationAngle=smiData.RigidTransform(58).angle  RotationArbitraryAxis=smiData.RigidTransform(58).axis  FollAlignAxisA=+X  BaseAlignAxisA=+Y  FollAlignAxisB=+Y  BaseAlignAxisB=+Z  RotationSequenceAxes=FollowerAxes  RotationSequence=XYX  RotationSequenceAngles=[0 0 0]  RotationSequenceAnglesUnits=deg  RotationMatrix=[1 0 0; 0 1 0; 0 0 1]
  Transform31 : sm_lib/Frames and Transforms/Rigid Transform  TranslationMethod=Cartesian  TranslationStandardOffset=0  TranslationLengthUnit=mm  TranslationStandardAxis=+Z  TranslationCartesianOffset=smiData.RigidTransform(59).translation  TranslationROffset=0  TranslationROffsetUnits=m  TranslationZOffset=0  TranslationZOffsetUnits=m  TranslationThetaOffset=0  TranslationThetaOffsetUnits=deg  RotationMethod=ArbitraryAxis  RotationAngleUnits=rad  RotationStandardAxis=+Z  RotationAngle=smiData.RigidTransform(59).angle  RotationArbitraryAxis=smiData.RigidTransform(59).axis  FollAlignAxisA=+X  BaseAlignAxisA=+Y  FollAlignAxisB=+Y  BaseAlignAxisB=+Z  RotationSequenceAxes=FollowerAxes  RotationSequence=XYX  RotationSequenceAngles=[0 0 0]  RotationSequenceAnglesUnits=deg  RotationMatrix=[1 0 0; 0 1 0; 0 0 1]
  Transform32 : sm_lib/Frames and Transforms/Rigid Transform  TranslationMethod=Cartesian  TranslationStandardOffset=0  TranslationLengthUnit=mm  TranslationStandardAxis=+Z  TranslationCartesianOffset=smiData.RigidTransform(60).translation  TranslationROffset=0  TranslationROffsetUnits=m  TranslationZOffset=0  TranslationZOffsetUnits=m  TranslationThetaOffset=0  TranslationThetaOffsetUnits=deg  RotationMethod=ArbitraryAxis  RotationAngleUnits=rad  RotationStandardAxis=+Z  RotationAngle=smiData.RigidTransform(60).angle  RotationArbitraryAxis=smiData.RigidTransform(60).axis  FollAlignAxisA=+X  BaseAlignAxisA=+Y  FollAlignAxisB=+Y  BaseAlignAxisB=+Z  RotationSequenceAxes=FollowerAxes  RotationSequence=XYX  RotationSequenceAngles=[0 0 0]  RotationSequenceAnglesUnits=deg  RotationMatrix=[1 0 0; 0 1 0; 0 0 1]
  Transform33 : sm_lib/Frames and Transforms/Rigid Transform  TranslationMethod=Cartesian  TranslationStandardOffset=0  TranslationLengthUnit=mm  TranslationStandardAxis=+Z  TranslationCartesianOffset=smiData.RigidTransform(61).translation  TranslationROffset=0  TranslationROffsetUnits=m  TranslationZOffset=0  TranslationZOffsetUnits=m  TranslationThetaOffset=0  TranslationThetaOffsetUnits=deg  RotationMethod=ArbitraryAxis  RotationAngleUnits=rad  RotationStandardAxis=+Z  RotationAngle=smiData.RigidTransform(61).angle  RotationArbitraryAxis=smiData.RigidTransform(61).axis  FollAlignAxisA=+X  BaseAlignAxisA=+Y  FollAlignAxisB=+Y  BaseAlignAxisB=+Z  RotationSequenceAxes=FollowerAxes  RotationSequence=XYX  RotationSequenceAngles=[0 0 0]  RotationSequenceAnglesUnits=deg  RotationMatrix=[1 0 0; 0 1 0; 0 0 1]
  Transform34 : sm_lib/Frames and Transforms/Rigid Transform  TranslationMethod=Cartesian  TranslationStandardOffset=0  TranslationLengthUnit=mm  TranslationStandardAxis=+Z  TranslationCartesianOffset=smiData.RigidTransform(62).translation  TranslationROffset=0  TranslationROffsetUnits=m  TranslationZOffset=0  TranslationZOffsetUnits=m  TranslationThetaOffset=0  TranslationThetaOffsetUnits=deg  RotationMethod=ArbitraryAxis  RotationAngleUnits=rad  RotationStandardAxis=+Z  RotationAngle=smiData.RigidTransform(62).angle  RotationArbitraryAxis=smiData.RigidTransform(62).axis  FollAlignAxisA=+X  BaseAlignAxisA=+Y  FollAlignAxisB=+Y  BaseAlignAxisB=+Z  RotationSequenceAxes=FollowerAxes  RotationSequence=XYX  RotationSequenceAngles=[0 0 0]  RotationSequenceAnglesUnits=deg  RotationMatrix=[1 0 0; 0 1 0; 0 0 1]
  Transform35 : sm_lib/Frames and Transforms/Rigid Transform  TranslationMethod=Cartesian  TranslationStandardOffset=0  TranslationLengthUnit=mm  TranslationStandardAxis=+Z  TranslationCartesianOffset=smiData.RigidTransform(63).translation  TranslationROffset=0  TranslationROffsetUnits=m  TranslationZOffset=0  TranslationZOffsetUnits=m  TranslationThetaOffset=0  TranslationThetaOffsetUnits=deg  RotationMethod=ArbitraryAxis  RotationAngleUnits=rad  RotationStandardAxis=+Z  RotationAngle=smiData.RigidTransform(63).angle  RotationArbitraryAxis=smiData.RigidTransform(63).axis  FollAlignAxisA=+X  BaseAlignAxisA=+Y  FollAlignAxisB=+Y  BaseAlignAxisB=+Z  RotationSequenceAxes=FollowerAxes  RotationSequence=XYX  RotationSequenceAngles=[0 0 0]  RotationSequenceAnglesUnits=deg  RotationMatrix=[1 0 0; 0 1 0; 0 0 1]
  Transform36 : sm_lib/Frames and Transforms/Rigid Transform  TranslationMethod=Cartesian  TranslationStandardOffset=0  TranslationLengthUnit=mm  TranslationStandardAxis=+Z  TranslationCartesianOffset=smiData.RigidTransform(64).translation  TranslationROffset=0  TranslationROffsetUnits=m  TranslationZOffset=0  TranslationZOffsetUnits=m  TranslationThetaOffset=0  TranslationThetaOffsetUnits=deg  RotationMethod=ArbitraryAxis  RotationAngleUnits=rad  RotationStandardAxis=+Z  RotationAngle=smiData.RigidTransform(64).angle  RotationArbitraryAxis=smiData.RigidTransform(64).axis  FollAlignAxisA=+X  BaseAlignAxisA=+Y  FollAlignAxisB=+Y  BaseAlignAxisB=+Z  RotationSequenceAxes=FollowerAxes  RotationSequence=XYX  RotationSequenceAngles=[0 0 0]  RotationSequenceAnglesUnits=deg  RotationMatrix=[1 0 0; 0 1 0; 0 0 1]
  Transform37 : sm_lib/Frames and Transforms/Rigid Transform  TranslationMethod=Cartesian  TranslationStandardOffset=0  TranslationLengthUnit=mm  TranslationStandardAxis=+Z  TranslationCartesianOffset=smiData.RigidTransform(65).translation  TranslationROffset=0  TranslationROffsetUnits=m  TranslationZOffset=0  TranslationZOffsetUnits=m  TranslationThetaOffset=0  TranslationThetaOffsetUnits=deg  RotationMethod=ArbitraryAxis  RotationAngleUnits=rad  RotationStandardAxis=+Z  RotationAngle=smiData.RigidTransform(65).angle  RotationArbitraryAxis=smiData.RigidTransform(65).axis  FollAlignAxisA=+X  BaseAlignAxisA=+Y  FollAlignAxisB=+Y  BaseAlignAxisB=+Z  RotationSequenceAxes=FollowerAxes  RotationSequence=XYX  RotationSequenceAngles=[0 0 0]  RotationSequenceAnglesUnits=deg  RotationMatrix=[1 0 0; 0 1 0; 0 0 1]
  Transform38 : sm_lib/Frames and Transforms/Rigid Transform  TranslationMethod=Cartesian  TranslationStandardOffset=0  TranslationLengthUnit=mm  TranslationStandardAxis=+Z  TranslationCartesianOffset=smiData.RigidTransform(66).translation  TranslationROffset=0  TranslationROffsetUnits=m  TranslationZOffset=0  TranslationZOffsetUnits=m  TranslationThetaOffset=0  TranslationThetaOffsetUnits=deg  RotationMethod=ArbitraryAxis  RotationAngleUnits=rad  RotationStandardAxis=+Z  RotationAngle=smiData.RigidTransform(66).angle  RotationArbitraryAxis=smiData.RigidTransform(66).axis  FollAlignAxisA=+X  BaseAlignAxisA=+Y  FollAlignAxisB=+Y  BaseAlignAxisB=+Z  RotationSequenceAxes=FollowerAxes  RotationSequence=XYX  RotationSequenceAngles=[0 0 0]  RotationSequenceAnglesUnits=deg  RotationMatrix=[1 0 0; 0 1 0; 0 0 1]
  Transform39 : sm_lib/Frames and Transforms/Rigid Transform  TranslationMethod=Cartesian  TranslationStandardOffset=0  TranslationLengthUnit=mm  TranslationStandardAxis=+Z  TranslationCartesianOffset=smiData.RigidTransform(67).translation  TranslationROffset=0  TranslationROffsetUnits=m  TranslationZOffset=0  TranslationZOffsetUnits=m  TranslationThetaOffset=0  TranslationThetaOffsetUnits=deg  RotationMethod=ArbitraryAxis  RotationAngleUnits=rad  RotationStandardAxis=+Z  RotationAngle=smiData.RigidTransform(67).angle  RotationArbitraryAxis=smiData.RigidTransform(67).axis  FollAlignAxisA=+X  BaseAlignAxisA=+Y  FollAlignAxisB=+Y  BaseAlignAxisB=+Z  RotationSequenceAxes=FollowerAxes  RotationSequence=XYX  RotationSequenceAngles=[0 0 0]  RotationSequenceAnglesUnits=deg  RotationMatrix=[1 0 0; 0 1 0; 0 0 1]
  Transform4 : sm_lib/Frames and Transforms/Rigid Transform  TranslationMethod=Cartesian  TranslationStandardOffset=0  TranslationLengthUnit=mm  TranslationStandardAxis=+Z  TranslationCartesianOffset=smiData.RigidTransform(32).translation  TranslationROffset=0  TranslationROffsetUnits=m  TranslationZOffset=0  TranslationZOffsetUnits=m  TranslationThetaOffset=0  TranslationThetaOffsetUnits=deg  RotationMethod=ArbitraryAxis  RotationAngleUnits=rad  RotationStandardAxis=+Z  RotationAngle=smiData.RigidTransform(32).angle  RotationArbitraryAxis=smiData.RigidTransform(32).axis  FollAlignAxisA=+X  BaseAlignAxisA=+Y  FollAlignAxisB=+Y  BaseAlignAxisB=+Z  RotationSequenceAxes=FollowerAxes  RotationSequence=XYX  RotationSequenceAngles=[0 0 0]  RotationSequenceAnglesUnits=deg  RotationMatrix=[1 0 0; 0 1 0; 0 0 1]
  Transform40 : sm_lib/Frames and Transforms/Rigid Transform  TranslationMethod=Cartesian  TranslationStandardOffset=0  TranslationLengthUnit=mm  TranslationStandardAxis=+Z  TranslationCartesianOffset=smiData.RigidTransform(68).translation  TranslationROffset=0  TranslationROffsetUnits=m  TranslationZOffset=0  TranslationZOffsetUnits=m  TranslationThetaOffset=0  TranslationThetaOffsetUnits=deg  RotationMethod=ArbitraryAxis  RotationAngleUnits=rad  RotationStandardAxis=+Z  RotationAngle=smiData.RigidTransform(68).angle  RotationArbitraryAxis=smiData.RigidTransform(68).axis  FollAlignAxisA=+X  BaseAlignAxisA=+Y  FollAlignAxisB=+Y  BaseAlignAxisB=+Z  RotationSequenceAxes=FollowerAxes  RotationSequence=XYX  RotationSequenceAngles=[0 0 0]  RotationSequenceAnglesUnits=deg  RotationMatrix=[1 0 0; 0 1 0; 0 0 1]
  Transform41 : sm_lib/Frames and Transforms/Rigid Transform  TranslationMethod=Cartesian  TranslationStandardOffset=0  TranslationLengthUnit=mm  TranslationStandardAxis=+Z  TranslationCartesianOffset=smiData.RigidTransform(69).translation  TranslationROffset=0  TranslationROffsetUnits=m  TranslationZOffset=0  TranslationZOffsetUnits=m  TranslationThetaOffset=0  TranslationThetaOffsetUnits=deg  RotationMethod=ArbitraryAxis  RotationAngleUnits=rad  RotationStandardAxis=+Z  RotationAngle=smiData.RigidTransform(69).angle  RotationArbitraryAxis=smiData.RigidTransform(69).axis  FollAlignAxisA=+X  BaseAlignAxisA=+Y  FollAlignAxisB=+Y  BaseAlignAxisB=+Z  RotationSequenceAxes=FollowerAxes  RotationSequence=XYX  RotationSequenceAngles=[0 0 0]  RotationSequenceAnglesUnits=deg  RotationMatrix=[1 0 0; 0 1 0; 0 0 1]
  Transform42 : sm_lib/Frames and Transforms/Rigid Transform  TranslationMethod=Cartesian  TranslationStandardOffset=0  TranslationLengthUnit=mm  TranslationStandardAxis=+Z  TranslationCartesianOffset=smiData.RigidTransform(70).translation  TranslationROffset=0  TranslationROffsetUnits=m  TranslationZOffset=0  TranslationZOffsetUnits=m  TranslationThetaOffset=0  TranslationThetaOffsetUnits=deg  RotationMethod=ArbitraryAxis  RotationAngleUnits=rad  RotationStandardAxis=+Z  RotationAngle=smiData.RigidTransform(70).angle  RotationArbitraryAxis=smiData.RigidTransform(70).axis  FollAlignAxisA=+X  BaseAlignAxisA=+Y  FollAlignAxisB=+Y  BaseAlignAxisB=+Z  RotationSequenceAxes=FollowerAxes  RotationSequence=XYX  RotationSequenceAngles=[0 0 0]  RotationSequenceAnglesUnits=deg  RotationMatrix=[1 0 0; 0 1 0; 0 0 1]
  Transform43 : sm_lib/Frames and Transforms/Rigid Transform  TranslationMethod=Cartesian  TranslationStandardOffset=0  TranslationLengthUnit=mm  TranslationStandardAxis=+Z  TranslationCartesianOffset=smiData.RigidTransform(71).translation  TranslationROffset=0  TranslationROffsetUnits=m  TranslationZOffset=0  TranslationZOffsetUnits=m  TranslationThetaOffset=0  TranslationThetaOffsetUnits=deg  RotationMethod=ArbitraryAxis  RotationAngleUnits=rad  RotationStandardAxis=+Z  RotationAngle=smiData.RigidTransform(71).angle  RotationArbitraryAxis=smiData.RigidTransform(71).axis  FollAlignAxisA=+X  BaseAlignAxisA=+Y  FollAlignAxisB=+Y  BaseAlignAxisB=+Z  RotationSequenceAxes=FollowerAxes  RotationSequence=XYX  RotationSequenceAngles=[0 0 0]  RotationSequenceAnglesUnits=deg  RotationMatrix=[1 0 0; 0 1 0; 0 0 1]
  Transform44 : sm_lib/Frames and Transforms/Rigid Transform  TranslationMethod=Cartesian  TranslationStandardOffset=0  TranslationLengthUnit=mm  TranslationStandardAxis=+Z  TranslationCartesianOffset=smiData.RigidTransform(72).translation  TranslationROffset=0  TranslationROffsetUnits=m  TranslationZOffset=0  TranslationZOffsetUnits=m  TranslationThetaOffset=0  TranslationThetaOffsetUnits=deg  RotationMethod=ArbitraryAxis  RotationAngleUnits=rad  RotationStandardAxis=+Z  RotationAngle=smiData.RigidTransform(72).angle  RotationArbitraryAxis=smiData.RigidTransform(72).axis  FollAlignAxisA=+X  BaseAlignAxisA=+Y  FollAlignAxisB=+Y  BaseAlignAxisB=+Z  RotationSequenceAxes=FollowerAxes  RotationSequence=XYX  RotationSequenceAngles=[0 0 0]  RotationSequenceAnglesUnits=deg  RotationMatrix=[1 0 0; 0 1 0; 0 0 1]
  Transform45 : sm_lib/Frames and Transforms/Rigid Transform  TranslationMethod=Cartesian  TranslationStandardOffset=0  TranslationLengthUnit=mm  TranslationStandardAxis=+Z  TranslationCartesianOffset=smiData.RigidTransform(73).translation  TranslationROffset=0  TranslationROffsetUnits=m  TranslationZOffset=0  TranslationZOffsetUnits=m  TranslationThetaOffset=0  TranslationThetaOffsetUnits=deg  RotationMethod=ArbitraryAxis  RotationAngleUnits=rad  RotationStandardAxis=+Z  RotationAngle=smiData.RigidTransform(73).angle  RotationArbitraryAxis=smiData.RigidTransform(73).axis  FollAlignAxisA=+X  BaseAlignAxisA=+Y  FollAlignAxisB=+Y  BaseAlignAxisB=+Z  RotationSequenceAxes=FollowerAxes  RotationSequence=XYX  RotationSequenceAngles=[0 0 0]  RotationSequenceAnglesUnits=deg  RotationMatrix=[1 0 0; 0 1 0; 0 0 1]
  Transform46 : sm_lib/Frames and Transforms/Rigid Transform  TranslationMethod=Cartesian  TranslationStandardOffset=0  TranslationLengthUnit=mm  TranslationStandardAxis=+Z  TranslationCartesianOffset=smiData.RigidTransform(74).translation  TranslationROffset=0  TranslationROffsetUnits=m  TranslationZOffset=0  TranslationZOffsetUnits=m  TranslationThetaOffset=0  TranslationThetaOffsetUnits=deg  RotationMethod=ArbitraryAxis  RotationAngleUnits=rad  RotationStandardAxis=+Z  RotationAngle=smiData.RigidTransform(74).angle  RotationArbitraryAxis=smiData.RigidTransform(74).axis  FollAlignAxisA=+X  BaseAlignAxisA=+Y  FollAlignAxisB=+Y  BaseAlignAxisB=+Z  RotationSequenceAxes=FollowerAxes  RotationSequence=XYX  RotationSequenceAngles=[0 0 0]  RotationSequenceAnglesUnits=deg  RotationMatrix=[1 0 0; 0 1 0; 0 0 1]
  Transform47 : sm_lib/Frames and Transforms/Rigid Transform  TranslationMethod=Cartesian  TranslationStandardOffset=0  TranslationLengthUnit=mm  TranslationStandardAxis=+Z  TranslationCartesianOffset=smiData.RigidTransform(75).translation  TranslationROffset=0  TranslationROffsetUnits=m  TranslationZOffset=0  TranslationZOffsetUnits=m  TranslationThetaOffset=0  TranslationThetaOffsetUnits=deg  RotationMethod=ArbitraryAxis  RotationAngleUnits=rad  RotationStandardAxis=+Z  RotationAngle=smiData.RigidTransform(75).angle  RotationArbitraryAxis=smiData.RigidTransform(75).axis  FollAlignAxisA=+X  BaseAlignAxisA=+Y  FollAlignAxisB=+Y  BaseAlignAxisB=+Z  RotationSequenceAxes=FollowerAxes  RotationSequence=XYX  RotationSequenceAngles=[0 0 0]  RotationSequenceAnglesUnits=deg  RotationMatrix=[1 0 0; 0 1 0; 0 0 1]
  Transform48 : sm_lib/Frames and Transforms/Rigid Transform  TranslationMethod=Cartesian  TranslationStandardOffset=0  TranslationLengthUnit=mm  TranslationStandardAxis=+Z  TranslationCartesianOffset=smiData.RigidTransform(76).translation  TranslationROffset=0  TranslationROffsetUnits=m  TranslationZOffset=0  TranslationZOffsetUnits=m  TranslationThetaOffset=0  TranslationThetaOffsetUnits=deg  RotationMethod=ArbitraryAxis  RotationAngleUnits=rad  RotationStandardAxis=+Z  RotationAngle=smiData.RigidTransform(76).angle  RotationArbitraryAxis=smiData.RigidTransform(76).axis  FollAlignAxisA=+X  BaseAlignAxisA=+Y  FollAlignAxisB=+Y  BaseAlignAxisB=+Z  RotationSequenceAxes=FollowerAxes  RotationSequence=XYX  RotationSequenceAngles=[0 0 0]  RotationSequenceAnglesUnits=deg  RotationMatrix=[1 0 0; 0 1 0; 0 0 1]
  Transform49 : sm_lib/Frames and Transforms/Rigid Transform  TranslationMethod=Cartesian  TranslationStandardOffset=0  TranslationLengthUnit=mm  TranslationStandardAxis=+Z  TranslationCartesianOffset=smiData.RigidTransform(77).translation  TranslationROffset=0  TranslationROffsetUnits=m  TranslationZOffset=0  TranslationZOffsetUnits=m  TranslationThetaOffset=0  TranslationThetaOffsetUnits=deg  RotationMethod=ArbitraryAxis  RotationAngleUnits=rad  RotationStandardAxis=+Z  RotationAngle=smiData.RigidTransform(77).angle  RotationArbitraryAxis=smiData.RigidTransform(77).axis  FollAlignAxisA=+X  BaseAlignAxisA=+Y  FollAlignAxisB=+Y  BaseAlignAxisB=+Z  RotationSequenceAxes=FollowerAxes  RotationSequence=XYX  RotationSequenceAngles=[0 0 0]  RotationSequenceAnglesUnits=deg  RotationMatrix=[1 0 0; 0 1 0; 0 0 1]
  Transform5 : sm_lib/Frames and Transforms/Rigid Transform  TranslationMethod=Cartesian  TranslationStandardOffset=0  TranslationLengthUnit=mm  TranslationStandardAxis=+Z  TranslationCartesianOffset=smiData.RigidTransform(33).translation  TranslationROffset=0  TranslationROffsetUnits=m  TranslationZOffset=0  TranslationZOffsetUnits=m  TranslationThetaOffset=0  TranslationThetaOffsetUnits=deg  RotationMethod=ArbitraryAxis  RotationAngleUnits=rad  RotationStandardAxis=+Z  RotationAngle=smiData.RigidTransform(33).angle  RotationArbitraryAxis=smiData.RigidTransform(33).axis  FollAlignAxisA=+X  BaseAlignAxisA=+Y  FollAlignAxisB=+Y  BaseAlignAxisB=+Z  RotationSequenceAxes=FollowerAxes  RotationSequence=XYX  RotationSequenceAngles=[0 0 0]  RotationSequenceAnglesUnits=deg  RotationMatrix=[1 0 0; 0 1 0; 0 0 1]
  Transform50 : sm_lib/Frames and Transforms/Rigid Transform  TranslationMethod=Cartesian  TranslationStandardOffset=0  TranslationLengthUnit=mm  TranslationStandardAxis=+Z  TranslationCartesianOffset=smiData.RigidTransform(78).translation  TranslationROffset=0  TranslationROffsetUnits=m  TranslationZOffset=0  TranslationZOffsetUnits=m  TranslationThetaOffset=0  TranslationThetaOffsetUnits=deg  RotationMethod=ArbitraryAxis  RotationAngleUnits=rad  RotationStandardAxis=+Z  RotationAngle=smiData.RigidTransform(78).angle  RotationArbitraryAxis=smiData.RigidTransform(78).axis  FollAlignAxisA=+X  BaseAlignAxisA=+Y  FollAlignAxisB=+Y  BaseAlignAxisB=+Z  RotationSequenceAxes=FollowerAxes  RotationSequence=XYX  RotationSequenceAngles=[0 0 0]  RotationSequenceAnglesUnits=deg  RotationMatrix=[1 0 0; 0 1 0; 0 0 1]
  Transform51 : sm_lib/Frames and Transforms/Rigid Transform  TranslationMethod=Cartesian  TranslationStandardOffset=0  TranslationLengthUnit=mm  TranslationStandardAxis=+Z  TranslationCartesianOffset=smiData.RigidTransform(79).translation  TranslationROffset=0  TranslationROffsetUnits=m  TranslationZOffset=0  TranslationZOffsetUnits=m  TranslationThetaOffset=0  TranslationThetaOffsetUnits=deg  RotationMethod=ArbitraryAxis  RotationAngleUnits=rad  RotationStandardAxis=+Z  RotationAngle=smiData.RigidTransform(79).angle  RotationArbitraryAxis=smiData.RigidTransform(79).axis  FollAlignAxisA=+X  BaseAlignAxisA=+Y  FollAlignAxisB=+Y  BaseAlignAxisB=+Z  RotationSequenceAxes=FollowerAxes  RotationSequence=XYX  RotationSequenceAngles=[0 0 0]  RotationSequenceAnglesUnits=deg  RotationMatrix=[1 0 0; 0 1 0; 0 0 1]
  Transform52 : sm_lib/Frames and Transforms/Rigid Transform  TranslationMethod=Cartesian  TranslationStandardOffset=0  TranslationLengthUnit=mm  TranslationStandardAxis=+Z  TranslationCartesianOffset=smiData.RigidTransform(80).translation  TranslationROffset=0  TranslationROffsetUnits=m  TranslationZOffset=0  TranslationZOffsetUnits=m  TranslationThetaOffset=0  TranslationThetaOffsetUnits=deg  RotationMethod=ArbitraryAxis  RotationAngleUnits=rad  RotationStandardAxis=+Z  RotationAngle=smiData.RigidTransform(80).angle  RotationArbitraryAxis=smiData.RigidTransform(80).axis  FollAlignAxisA=+X  BaseAlignAxisA=+Y  FollAlignAxisB=+Y  BaseAlignAxisB=+Z  RotationSequenceAxes=FollowerAxes  RotationSequence=XYX  RotationSequenceAngles=[0 0 0]  RotationSequenceAnglesUnits=deg  RotationMatrix=[1 0 0; 0 1 0; 0 0 1]
  Transform53 : sm_lib/Frames and Transforms/Rigid Transform  TranslationMethod=Cartesian  TranslationStandardOffset=0  TranslationLengthUnit=mm  TranslationStandardAxis=+Z  TranslationCartesianOffset=smiData.RigidTransform(81).translation  TranslationROffset=0  TranslationROffsetUnits=m  TranslationZOffset=0  TranslationZOffsetUnits=m  TranslationThetaOffset=0  TranslationThetaOffsetUnits=deg  RotationMethod=ArbitraryAxis  RotationAngleUnits=rad  RotationStandardAxis=+Z  RotationAngle=smiData.RigidTransform(81).angle  RotationArbitraryAxis=smiData.RigidTransform(81).axis  FollAlignAxisA=+X  BaseAlignAxisA=+Y  FollAlignAxisB=+Y  BaseAlignAxisB=+Z  RotationSequenceAxes=FollowerAxes  RotationSequence=XYX  RotationSequenceAngles=[0 0 0]  RotationSequenceAnglesUnits=deg  RotationMatrix=[1 0 0; 0 1 0; 0 0 1]
  Transform54 : sm_lib/Frames and Transforms/Rigid Transform  TranslationMethod=Cartesian  TranslationStandardOffset=0  TranslationLengthUnit=mm  TranslationStandardAxis=+Z  TranslationCartesianOffset=smiData.RigidTransform(82).translation  TranslationROffset=0  TranslationROffsetUnits=m  TranslationZOffset=0  TranslationZOffsetUnits=m  TranslationThetaOffset=0  TranslationThetaOffsetUnits=deg  RotationMethod=ArbitraryAxis  RotationAngleUnits=rad  RotationStandardAxis=+Z  RotationAngle=smiData.RigidTransform(82).angle  RotationArbitraryAxis=smiData.RigidTransform(82).axis  FollAlignAxisA=+X  BaseAlignAxisA=+Y  FollAlignAxisB=+Y  BaseAlignAxisB=+Z  RotationSequenceAxes=FollowerAxes  RotationSequence=XYX  RotationSequenceAngles=[0 0 0]  RotationSequenceAnglesUnits=deg  RotationMatrix=[1 0 0; 0 1 0; 0 0 1]
  Transform55 : sm_lib/Frames and Transforms/Rigid Transform  TranslationMethod=Cartesian  TranslationStandardOffset=0  TranslationLengthUnit=mm  TranslationStandardAxis=+Z  TranslationCartesianOffset=smiData.RigidTransform(83).translation  TranslationROffset=0  TranslationROffsetUnits=m  TranslationZOffset=0  TranslationZOffsetUnits=m  TranslationThetaOffset=0  TranslationThetaOffsetUnits=deg  RotationMethod=ArbitraryAxis  RotationAngleUnits=rad  RotationStandardAxis=+Z  RotationAngle=smiData.RigidTransform(83).angle  RotationArbitraryAxis=smiData.RigidTransform(83).axis  FollAlignAxisA=+X  BaseAlignAxisA=+Y  FollAlignAxisB=+Y  BaseAlignAxisB=+Z  RotationSequenceAxes=FollowerAxes  RotationSequence=XYX  RotationSequenceAngles=[0 0 0]  RotationSequenceAnglesUnits=deg  RotationMatrix=[1 0 0; 0 1 0; 0 0 1]
  Transform56 : sm_lib/Frames and Transforms/Rigid Transform  TranslationMethod=Cartesian  TranslationStandardOffset=0  TranslationLengthUnit=mm  TranslationStandardAxis=+Z  TranslationCartesianOffset=smiData.RigidTransform(84).translation  TranslationROffset=0  TranslationROffsetUnits=m  TranslationZOffset=0  TranslationZOffsetUnits=m  TranslationThetaOffset=0  TranslationThetaOffsetUnits=deg  RotationMethod=ArbitraryAxis  RotationAngleUnits=rad  RotationStandardAxis=+Z  RotationAngle=smiData.RigidTransform(84).angle  RotationArbitraryAxis=smiData.RigidTransform(84).axis  FollAlignAxisA=+X  BaseAlignAxisA=+Y  FollAlignAxisB=+Y  BaseAlignAxisB=+Z  RotationSequenceAxes=FollowerAxes  RotationSequence=XYX  RotationSequenceAngles=[0 0 0]  RotationSequenceAnglesUnits=deg  RotationMatrix=[1 0 0; 0 1 0; 0 0 1]
  Transform57 : sm_lib/Frames and Transforms/Rigid Transform  TranslationMethod=Cartesian  TranslationStandardOffset=0  TranslationLengthUnit=mm  TranslationStandardAxis=+Z  TranslationCartesianOffset=smiData.RigidTransform(85).translation  TranslationROffset=0  TranslationROffsetUnits=m  TranslationZOffset=0  TranslationZOffsetUnits=m  TranslationThetaOffset=0  TranslationThetaOffsetUnits=deg  RotationMethod=ArbitraryAxis  RotationAngleUnits=rad  RotationStandardAxis=+Z  RotationAngle=smiData.RigidTransform(85).angle  RotationArbitraryAxis=smiData.RigidTransform(85).axis  FollAlignAxisA=+X  BaseAlignAxisA=+Y  FollAlignAxisB=+Y  BaseAlignAxisB=+Z  RotationSequenceAxes=FollowerAxes  RotationSequence=XYX  RotationSequenceAngles=[0 0 0]  RotationSequenceAnglesUnits=deg  RotationMatrix=[1 0 0; 0 1 0; 0 0 1]
  Transform58 : sm_lib/Frames and Transforms/Rigid Transform  TranslationMethod=Cartesian  TranslationStandardOffset=0  TranslationLengthUnit=mm  TranslationStandardAxis=+Z  TranslationCartesianOffset=smiData.RigidTransform(86).translation  TranslationROffset=0  TranslationROffsetUnits=m  TranslationZOffset=0  TranslationZOffsetUnits=m  TranslationThetaOffset=0  TranslationThetaOffsetUnits=deg  RotationMethod=ArbitraryAxis  RotationAngleUnits=rad  RotationStandardAxis=+Z  RotationAngle=smiData.RigidTransform(86).angle  RotationArbitraryAxis=smiData.RigidTransform(86).axis  FollAlignAxisA=+X  BaseAlignAxisA=+Y  FollAlignAxisB=+Y  BaseAlignAxisB=+Z  RotationSequenceAxes=FollowerAxes  RotationSequence=XYX  RotationSequenceAngles=[0 0 0]  RotationSequenceAnglesUnits=deg  RotationMatrix=[1 0 0; 0 1 0; 0 0 1]
  Transform59 : sm_lib/Frames and Transforms/Rigid Transform  TranslationMethod=Cartesian  TranslationStandardOffset=0  TranslationLengthUnit=mm  TranslationStandardAxis=+Z  TranslationCartesianOffset=smiData.RigidTransform(87).translation  TranslationROffset=0  TranslationROffsetUnits=m  TranslationZOffset=0  TranslationZOffsetUnits=m  TranslationThetaOffset=0  TranslationThetaOffsetUnits=deg  RotationMethod=ArbitraryAxis  RotationAngleUnits=rad  RotationStandardAxis=+Z  RotationAngle=smiData.RigidTransform(87).angle  RotationArbitraryAxis=smiData.RigidTransform(87).axis  FollAlignAxisA=+X  BaseAlignAxisA=+Y  FollAlignAxisB=+Y  BaseAlignAxisB=+Z  RotationSequenceAxes=FollowerAxes  RotationSequence=XYX  RotationSequenceAngles=[0 0 0]  RotationSequenceAnglesUnits=deg  RotationMatrix=[1 0 0; 0 1 0; 0 0 1]
  Transform6 : sm_lib/Frames and Transforms/Rigid Transform  TranslationMethod=Cartesian  TranslationStandardOffset=0  TranslationLengthUnit=mm  TranslationStandardAxis=+Z  TranslationCartesianOffset=smiData.RigidTransform(34).translation  TranslationROffset=0  TranslationROffsetUnits=m  TranslationZOffset=0  TranslationZOffsetUnits=m  TranslationThetaOffset=0  TranslationThetaOffsetUnits=deg  RotationMethod=ArbitraryAxis  RotationAngleUnits=rad  RotationStandardAxis=+Z  RotationAngle=smiData.RigidTransform(34).angle  RotationArbitraryAxis=smiData.RigidTransform(34).axis  FollAlignAxisA=+X  BaseAlignAxisA=+Y  FollAlignAxisB=+Y  BaseAlignAxisB=+Z  RotationSequenceAxes=FollowerAxes  RotationSequence=XYX  RotationSequenceAngles=[0 0 0]  RotationSequenceAnglesUnits=deg  RotationMatrix=[1 0 0; 0 1 0; 0 0 1]
  Transform60 : sm_lib/Frames and Transforms/Rigid Transform  TranslationMethod=Cartesian  TranslationStandardOffset=0  TranslationLengthUnit=mm  TranslationStandardAxis=+Z  TranslationCartesianOffset=smiData.RigidTransform(88).translation  TranslationROffset=0  TranslationROffsetUnits=m  TranslationZOffset=0  TranslationZOffsetUnits=m  TranslationThetaOffset=0  TranslationThetaOffsetUnits=deg  RotationMethod=ArbitraryAxis  RotationAngleUnits=rad  RotationStandardAxis=+Z  RotationAngle=smiData.RigidTransform(88).angle  RotationArbitraryAxis=smiData.RigidTransform(88).axis  FollAlignAxisA=+X  BaseAlignAxisA=+Y  FollAlignAxisB=+Y  BaseAlignAxisB=+Z  RotationSequenceAxes=FollowerAxes  RotationSequence=XYX  RotationSequenceAngles=[0 0 0]  RotationSequenceAnglesUnits=deg  RotationMatrix=[1 0 0; 0 1 0; 0 0 1]
  Transform61 : sm_lib/Frames and Transforms/Rigid Transform  TranslationMethod=Cartesian  TranslationStandardOffset=0  TranslationLengthUnit=mm  TranslationStandardAxis=+Z  TranslationCartesianOffset=smiData.RigidTransform(89).translation  TranslationROffset=0  TranslationROffsetUnits=m  TranslationZOffset=0  TranslationZOffsetUnits=m  TranslationThetaOffset=0  TranslationThetaOffsetUnits=deg  RotationMethod=ArbitraryAxis  RotationAngleUnits=rad  RotationStandardAxis=+Z  RotationAngle=smiData.RigidTransform(89).angle  RotationArbitraryAxis=smiData.RigidTransform(89).axis  FollAlignAxisA=+X  BaseAlignAxisA=+Y  FollAlignAxisB=+Y  BaseAlignAxisB=+Z  RotationSequenceAxes=FollowerAxes  RotationSequence=XYX  RotationSequenceAngles=[0 0 0]  RotationSequenceAnglesUnits=deg  RotationMatrix=[1 0 0; 0 1 0; 0 0 1]
  Transform62 : sm_lib/Frames and Transforms/Rigid Transform  TranslationMethod=Cartesian  TranslationStandardOffset=0  TranslationLengthUnit=mm  TranslationStandardAxis=+Z  TranslationCartesianOffset=smiData.RigidTransform(90).translation  TranslationROffset=0  TranslationROffsetUnits=m  TranslationZOffset=0  TranslationZOffsetUnits=m  TranslationThetaOffset=0  TranslationThetaOffsetUnits=deg  RotationMethod=ArbitraryAxis  RotationAngleUnits=rad  RotationStandardAxis=+Z  RotationAngle=smiData.RigidTransform(90).angle  RotationArbitraryAxis=smiData.RigidTransform(90).axis  FollAlignAxisA=+X  BaseAlignAxisA=+Y  FollAlignAxisB=+Y  BaseAlignAxisB=+Z  RotationSequenceAxes=FollowerAxes  RotationSequence=XYX  RotationSequenceAngles=[0 0 0]  RotationSequenceAnglesUnits=deg  RotationMatrix=[1 0 0; 0 1 0; 0 0 1]
  Transform63 : sm_lib/Frames and Transforms/Rigid Transform  TranslationMethod=Cartesian  TranslationStandardOffset=0  TranslationLengthUnit=mm  TranslationStandardAxis=+Z  TranslationCartesianOffset=smiData.RigidTransform(91).translation  TranslationROffset=0  TranslationROffsetUnits=m  TranslationZOffset=0  TranslationZOffsetUnits=m  TranslationThetaOffset=0  TranslationThetaOffsetUnits=deg  RotationMethod=ArbitraryAxis  RotationAngleUnits=rad  RotationStandardAxis=+Z  RotationAngle=smiData.RigidTransform(91).angle  RotationArbitraryAxis=smiData.RigidTransform(91).axis  FollAlignAxisA=+X  BaseAlignAxisA=+Y  FollAlignAxisB=+Y  BaseAlignAxisB=+Z  RotationSequenceAxes=FollowerAxes  RotationSequence=XYX  RotationSequenceAngles=[0 0 0]  RotationSequenceAnglesUnits=deg  RotationMatrix=[1 0 0; 0 1 0; 0 0 1]
  Transform64 : sm_lib/Frames and Transforms/Rigid Transform  TranslationMethod=Cartesian  TranslationStandardOffset=0  TranslationLengthUnit=mm  TranslationStandardAxis=+Z  TranslationCartesianOffset=smiData.RigidTransform(92).translation  TranslationROffset=0  TranslationROffsetUnits=m  TranslationZOffset=0  TranslationZOffsetUnits=m  TranslationThetaOffset=0  TranslationThetaOffsetUnits=deg  RotationMethod=ArbitraryAxis  RotationAngleUnits=rad  RotationStandardAxis=+Z  RotationAngle=smiData.RigidTransform(92).angle  RotationArbitraryAxis=smiData.RigidTransform(92).axis  FollAlignAxisA=+X  BaseAlignAxisA=+Y  FollAlignAxisB=+Y  BaseAlignAxisB=+Z  RotationSequenceAxes=FollowerAxes  RotationSequence=XYX  RotationSequenceAngles=[0 0 0]  RotationSequenceAnglesUnits=deg  RotationMatrix=[1 0 0; 0 1 0; 0 0 1]
  Transform65 : sm_lib/Frames and Transforms/Rigid Transform  TranslationMethod=Cartesian  TranslationStandardOffset=0  TranslationLengthUnit=mm  TranslationStandardAxis=+Z  TranslationCartesianOffset=smiData.RigidTransform(93).translation  TranslationROffset=0  TranslationROffsetUnits=m  TranslationZOffset=0  TranslationZOffsetUnits=m  TranslationThetaOffset=0  TranslationThetaOffsetUnits=deg  RotationMethod=ArbitraryAxis  RotationAngleUnits=rad  RotationStandardAxis=+Z  RotationAngle=smiData.RigidTransform(93).angle  RotationArbitraryAxis=smiData.RigidTransform(93).axis  FollAlignAxisA=+X  BaseAlignAxisA=+Y  FollAlignAxisB=+Y  BaseAlignAxisB=+Z  RotationSequenceAxes=FollowerAxes  RotationSequence=XYX  RotationSequenceAngles=[0 0 0]  RotationSequenceAnglesUnits=deg  RotationMatrix=[1 0 0; 0 1 0; 0 0 1]
  Transform66 : sm_lib/Frames and Transforms/Rigid Transform  TranslationMethod=Cartesian  TranslationStandardOffset=0  TranslationLengthUnit=mm  TranslationStandardAxis=+Z  TranslationCartesianOffset=smiData.RigidTransform(94).translation  TranslationROffset=0  TranslationROffsetUnits=m  TranslationZOffset=0  TranslationZOffsetUnits=m  TranslationThetaOffset=0  TranslationThetaOffsetUnits=deg  RotationMethod=ArbitraryAxis  RotationAngleUnits=rad  RotationStandardAxis=+Z  RotationAngle=smiData.RigidTransform(94).angle  RotationArbitraryAxis=smiData.RigidTransform(94).axis  FollAlignAxisA=+X  BaseAlignAxisA=+Y  FollAlignAxisB=+Y  BaseAlignAxisB=+Z  RotationSequenceAxes=FollowerAxes  RotationSequence=XYX  RotationSequenceAngles=[0 0 0]  RotationSequenceAnglesUnits=deg  RotationMatrix=[1 0 0; 0 1 0; 0 0 1]
  Transform67 : sm_lib/Frames and Transforms/Rigid Transform  TranslationMethod=Cartesian  TranslationStandardOffset=0  TranslationLengthUnit=mm  TranslationStandardAxis=+Z  TranslationCartesianOffset=smiData.RigidTransform(95).translation  TranslationROffset=0  TranslationROffsetUnits=m  TranslationZOffset=0  TranslationZOffsetUnits=m  TranslationThetaOffset=0  TranslationThetaOffsetUnits=deg  RotationMethod=ArbitraryAxis  RotationAngleUnits=rad  RotationStandardAxis=+Z  RotationAngle=smiData.RigidTransform(95).angle  RotationArbitraryAxis=smiData.RigidTransform(95).axis  FollAlignAxisA=+X  BaseAlignAxisA=+Y  FollAlignAxisB=+Y  BaseAlignAxisB=+Z  RotationSequenceAxes=FollowerAxes  RotationSequence=XYX  RotationSequenceAngles=[0 0 0]  RotationSequenceAnglesUnits=deg  RotationMatrix=[1 0 0; 0 1 0; 0 0 1]
  Transform68 : sm_lib/Frames and Transforms/Rigid Transform  TranslationMethod=Cartesian  TranslationStandardOffset=0  TranslationLengthUnit=mm  TranslationStandardAxis=+Z  TranslationCartesianOffset=smiData.RigidTransform(96).translation  TranslationROffset=0  TranslationROffsetUnits=m  TranslationZOffset=0  TranslationZOffsetUnits=m  TranslationThetaOffset=0  TranslationThetaOffsetUnits=deg  RotationMethod=ArbitraryAxis  RotationAngleUnits=rad  RotationStandardAxis=+Z  RotationAngle=smiData.RigidTransform(96).angle  RotationArbitraryAxis=smiData.RigidTransform(96).axis  FollAlignAxisA=+X  BaseAlignAxisA=+Y  FollAlignAxisB=+Y  BaseAlignAxisB=+Z  RotationSequenceAxes=FollowerAxes  RotationSequence=XYX  RotationSequenceAngles=[0 0 0]  RotationSequenceAnglesUnits=deg  RotationMatrix=[1 0 0; 0 1 0; 0 0 1]
  Transform69 : sm_lib/Frames and Transforms/Rigid Transform  TranslationMethod=Cartesian  TranslationStandardOffset=0  TranslationLengthUnit=mm  TranslationStandardAxis=+Z  TranslationCartesianOffset=smiData.RigidTransform(97).translation  TranslationROffset=0  TranslationROffsetUnits=m  TranslationZOffset=0  TranslationZOffsetUnits=m  TranslationThetaOffset=0  TranslationThetaOffsetUnits=deg  RotationMethod=ArbitraryAxis  RotationAngleUnits=rad  RotationStandardAxis=+Z  RotationAngle=smiData.RigidTransform(97).angle  RotationArbitraryAxis=smiData.RigidTransform(97).axis  FollAlignAxisA=+X  BaseAlignAxisA=+Y  FollAlignAxisB=+Y  BaseAlignAxisB=+Z  RotationSequenceAxes=FollowerAxes  RotationSequence=XYX  RotationSequenceAngles=[0 0 0]  RotationSequenceAnglesUnits=deg  RotationMatrix=[1 0 0; 0 1 0; 0 0 1]
  Transform7 : sm_lib/Frames and Transforms/Rigid Transform  TranslationMethod=Cartesian  TranslationStandardOffset=0  TranslationLengthUnit=mm  TranslationStandardAxis=+Z  TranslationCartesianOffset=smiData.RigidTransform(35).translation  TranslationROffset=0  TranslationROffsetUnits=m  TranslationZOffset=0  TranslationZOffsetUnits=m  TranslationThetaOffset=0  TranslationThetaOffsetUnits=deg  RotationMethod=ArbitraryAxis  RotationAngleUnits=rad  RotationStandardAxis=+Z  RotationAngle=smiData.RigidTransform(35).angle  RotationArbitraryAxis=smiData.RigidTransform(35).axis  FollAlignAxisA=+X  BaseAlignAxisA=+Y  FollAlignAxisB=+Y  BaseAlignAxisB=+Z  RotationSequenceAxes=FollowerAxes  RotationSequence=XYX  RotationSequenceAngles=[0 0 0]  RotationSequenceAnglesUnits=deg  RotationMatrix=[1 0 0; 0 1 0; 0 0 1]
  Transform70 : sm_lib/Frames and Transforms/Rigid Transform  TranslationMethod=Cartesian  TranslationStandardOffset=0  TranslationLengthUnit=mm  TranslationStandardAxis=+Z  TranslationCartesianOffset=smiData.RigidTransform(98).translation  TranslationROffset=0  TranslationROffsetUnits=m  TranslationZOffset=0  TranslationZOffsetUnits=m  TranslationThetaOffset=0  TranslationThetaOffsetUnits=deg  RotationMethod=ArbitraryAxis  RotationAngleUnits=rad  RotationStandardAxis=+Z  RotationAngle=smiData.RigidTransform(98).angle  RotationArbitraryAxis=smiData.RigidTransform(98).axis  FollAlignAxisA=+X  BaseAlignAxisA=+Y  FollAlignAxisB=+Y  BaseAlignAxisB=+Z  RotationSequenceAxes=FollowerAxes  RotationSequence=XYX  RotationSequenceAngles=[0 0 0]  RotationSequenceAnglesUnits=deg  RotationMatrix=[1 0 0; 0 1 0; 0 0 1]
  Transform71 : sm_lib/Frames and Transforms/Rigid Transform  TranslationMethod=Cartesian  TranslationStandardOffset=0  TranslationLengthUnit=mm  TranslationStandardAxis=+Z  TranslationCartesianOffset=smiData.RigidTransform(99).translation  TranslationROffset=0  TranslationROffsetUnits=m  TranslationZOffset=0  TranslationZOffsetUnits=m  TranslationThetaOffset=0  TranslationThetaOffsetUnits=deg  RotationMethod=ArbitraryAxis  RotationAngleUnits=rad  RotationStandardAxis=+Z  RotationAngle=smiData.RigidTransform(99).angle  RotationArbitraryAxis=smiData.RigidTransform(99).axis  FollAlignAxisA=+X  BaseAlignAxisA=+Y  FollAlignAxisB=+Y  BaseAlignAxisB=+Z  RotationSequenceAxes=FollowerAxes  RotationSequence=XYX  RotationSequenceAngles=[0 0 0]  RotationSequenceAnglesUnits=deg  RotationMatrix=[1 0 0; 0 1 0; 0 0 1]
  Transform72 : sm_lib/Frames and Transforms/Rigid Transform  TranslationMethod=Cartesian  TranslationStandardOffset=0  TranslationLengthUnit=mm  TranslationStandardAxis=+Z  TranslationCartesianOffset=smiData.RigidTransform(100).translation  TranslationROffset=0  TranslationROffsetUnits=m  TranslationZOffset=0  TranslationZOffsetUnits=m  TranslationThetaOffset=0  TranslationThetaOffsetUnits=deg  RotationMethod=ArbitraryAxis  RotationAngleUnits=rad  RotationStandardAxis=+Z  RotationAngle=smiData.RigidTransform(100).angle  RotationArbitraryAxis=smiData.RigidTransform(100).axis  FollAlignAxisA=+X  BaseAlignAxisA=+Y  FollAlignAxisB=+Y  BaseAlignAxisB=+Z  RotationSequenceAxes=FollowerAxes  RotationSequence=XYX  RotationSequenceAngles=[0 0 0]  RotationSequenceAnglesUnits=deg  RotationMatrix=[1 0 0; 0 1 0; 0 0 1]
  Transform73 : sm_lib/Frames and Transforms/Rigid Transform  TranslationMethod=Cartesian  TranslationStandardOffset=0  TranslationLengthUnit=mm  TranslationStandardAxis=+Z  TranslationCartesianOffset=smiData.RigidTransform(101).translation  TranslationROffset=0  TranslationROffsetUnits=m  TranslationZOffset=0  TranslationZOffsetUnits=m  TranslationThetaOffset=0  TranslationThetaOffsetUnits=deg  RotationMethod=ArbitraryAxis  RotationAngleUnits=rad  RotationStandardAxis=+Z  RotationAngle=smiData.RigidTransform(101).angle  RotationArbitraryAxis=smiData.RigidTransform(101).axis  FollAlignAxisA=+X  BaseAlignAxisA=+Y  FollAlignAxisB=+Y  BaseAlignAxisB=+Z  RotationSequenceAxes=FollowerAxes  RotationSequence=XYX  RotationSequenceAngles=[0 0 0]  RotationSequenceAnglesUnits=deg  RotationMatrix=[1 0 0; 0 1 0; 0 0 1]
  Transform74 : sm_lib/Frames and Transforms/Rigid Transform  TranslationMethod=Cartesian  TranslationStandardOffset=0  TranslationLengthUnit=mm  TranslationStandardAxis=+Z  TranslationCartesianOffset=smiData.RigidTransform(102).translation  TranslationROffset=0  TranslationROffsetUnits=m  TranslationZOffset=0  TranslationZOffsetUnits=m  TranslationThetaOffset=0  TranslationThetaOffsetUnits=deg  RotationMethod=ArbitraryAxis  RotationAngleUnits=rad  RotationStandardAxis=+Z  RotationAngle=smiData.RigidTransform(102).angle  RotationArbitraryAxis=smiData.RigidTransform(102).axis  FollAlignAxisA=+X  BaseAlignAxisA=+Y  FollAlignAxisB=+Y  BaseAlignAxisB=+Z  RotationSequenceAxes=FollowerAxes  RotationSequence=XYX  RotationSequenceAngles=[0 0 0]  RotationSequenceAnglesUnits=deg  RotationMatrix=[1 0 0; 0 1 0; 0 0 1]
  Transform75 : sm_lib/Frames and Transforms/Rigid Transform  TranslationMethod=Cartesian  TranslationStandardOffset=0  TranslationLengthUnit=mm  TranslationStandardAxis=+Z  TranslationCartesianOffset=smiData.RigidTransform(103).translation  TranslationROffset=0  TranslationROffsetUnits=m  TranslationZOffset=0  TranslationZOffsetUnits=m  TranslationThetaOffset=0  TranslationThetaOffsetUnits=deg  RotationMethod=ArbitraryAxis  RotationAngleUnits=rad  RotationStandardAxis=+Z  RotationAngle=smiData.RigidTransform(103).angle  RotationArbitraryAxis=smiData.RigidTransform(103).axis  FollAlignAxisA=+X  BaseAlignAxisA=+Y  FollAlignAxisB=+Y  BaseAlignAxisB=+Z  RotationSequenceAxes=FollowerAxes  RotationSequence=XYX  RotationSequenceAngles=[0 0 0]  RotationSequenceAnglesUnits=deg  RotationMatrix=[1 0 0; 0 1 0; 0 0 1]
  Transform76 : sm_lib/Frames and Transforms/Rigid Transform  TranslationMethod=Cartesian  TranslationStandardOffset=0  TranslationLengthUnit=mm  TranslationStandardAxis=+Z  TranslationCartesianOffset=smiData.RigidTransform(104).translation  TranslationROffset=0  TranslationROffsetUnits=m  TranslationZOffset=0  TranslationZOffsetUnits=m  TranslationThetaOffset=0  TranslationThetaOffsetUnits=deg  RotationMethod=ArbitraryAxis  RotationAngleUnits=rad  RotationStandardAxis=+Z  RotationAngle=smiData.RigidTransform(104).angle  RotationArbitraryAxis=smiData.RigidTransform(104).axis  FollAlignAxisA=+X  BaseAlignAxisA=+Y  FollAlignAxisB=+Y  BaseAlignAxisB=+Z  RotationSequenceAxes=FollowerAxes  RotationSequence=XYX  RotationSequenceAngles=[0 0 0]  RotationSequenceAnglesUnits=deg  RotationMatrix=[1 0 0; 0 1 0; 0 0 1]
  Transform77 : sm_lib/Frames and Transforms/Rigid Transform  TranslationMethod=Cartesian  TranslationStandardOffset=0  TranslationLengthUnit=mm  TranslationStandardAxis=+Z  TranslationCartesianOffset=smiData.RigidTransform(105).translation  TranslationROffset=0  TranslationROffsetUnits=m  TranslationZOffset=0  TranslationZOffsetUnits=m  TranslationThetaOffset=0  TranslationThetaOffsetUnits=deg  RotationMethod=ArbitraryAxis  RotationAngleUnits=rad  RotationStandardAxis=+Z  RotationAngle=smiData.RigidTransform(105).angle  RotationArbitraryAxis=smiData.RigidTransform(105).axis  FollAlignAxisA=+X  BaseAlignAxisA=+Y  FollAlignAxisB=+Y  BaseAlignAxisB=+Z  RotationSequenceAxes=FollowerAxes  RotationSequence=XYX  RotationSequenceAngles=[0 0 0]  RotationSequenceAnglesUnits=deg  RotationMatrix=[1 0 0; 0 1 0; 0 0 1]
  Transform78 : sm_lib/Frames and Transforms/Rigid Transform  TranslationMethod=Cartesian  TranslationStandardOffset=0  TranslationLengthUnit=mm  TranslationStandardAxis=+Z  TranslationCartesianOffset=smiData.RigidTransform(106).translation  TranslationROffset=0  TranslationROffsetUnits=m  TranslationZOffset=0  TranslationZOffsetUnits=m  TranslationThetaOffset=0  TranslationThetaOffsetUnits=deg  RotationMethod=ArbitraryAxis  RotationAngleUnits=rad  RotationStandardAxis=+Z  RotationAngle=smiData.RigidTransform(106).angle  RotationArbitraryAxis=smiData.RigidTransform(106).axis  FollAlignAxisA=+X  BaseAlignAxisA=+Y  FollAlignAxisB=+Y  BaseAlignAxisB=+Z  RotationSequenceAxes=FollowerAxes  RotationSequence=XYX  RotationSequenceAngles=[0 0 0]  RotationSequenceAnglesUnits=deg  RotationMatrix=[1 0 0; 0 1 0; 0 0 1]
  Transform79 : sm_lib/Frames and Transforms/Rigid Transform  TranslationMethod=Cartesian  TranslationStandardOffset=0  TranslationLengthUnit=mm  TranslationStandardAxis=+Z  TranslationCartesianOffset=smiData.RigidTransform(107).translation  TranslationROffset=0  TranslationROffsetUnits=m  TranslationZOffset=0  TranslationZOffsetUnits=m  TranslationThetaOffset=0  TranslationThetaOffsetUnits=deg  RotationMethod=ArbitraryAxis  RotationAngleUnits=rad  RotationStandardAxis=+Z  RotationAngle=smiData.RigidTransform(107).angle  RotationArbitraryAxis=smiData.RigidTransform(107).axis  FollAlignAxisA=+X  BaseAlignAxisA=+Y  FollAlignAxisB=+Y  BaseAlignAxisB=+Z  RotationSequenceAxes=FollowerAxes  RotationSequence=XYX  RotationSequenceAngles=[0 0 0]  RotationSequenceAnglesUnits=deg  RotationMatrix=[1 0 0; 0 1 0; 0 0 1]
  Transform8 : sm_lib/Frames and Transforms/Rigid Transform  TranslationMethod=Cartesian  TranslationStandardOffset=0  TranslationLengthUnit=mm  TranslationStandardAxis=+Z  TranslationCartesianOffset=smiData.RigidTransform(36).translation  TranslationROffset=0  TranslationROffsetUnits=m  TranslationZOffset=0  TranslationZOffsetUnits=m  TranslationThetaOffset=0  TranslationThetaOffsetUnits=deg  RotationMethod=ArbitraryAxis  RotationAngleUnits=rad  RotationStandardAxis=+Z  RotationAngle=smiData.RigidTransform(36).angle  RotationArbitraryAxis=smiData.RigidTransform(36).axis  FollAlignAxisA=+X  BaseAlignAxisA=+Y  FollAlignAxisB=+Y  BaseAlignAxisB=+Z  RotationSequenceAxes=FollowerAxes  RotationSequence=XYX  RotationSequenceAngles=[0 0 0]  RotationSequenceAnglesUnits=deg  RotationMatrix=[1 0 0; 0 1 0; 0 0 1]
  Transform80 : sm_lib/Frames and Transforms/Rigid Transform  TranslationMethod=Cartesian  TranslationStandardOffset=0  TranslationLengthUnit=mm  TranslationStandardAxis=+Z  TranslationCartesianOffset=smiData.RigidTransform(108).translation  TranslationROffset=0  TranslationROffsetUnits=m  TranslationZOffset=0  TranslationZOffsetUnits=m  TranslationThetaOffset=0  TranslationThetaOffsetUnits=deg  RotationMethod=ArbitraryAxis  RotationAngleUnits=rad  RotationStandardAxis=+Z  RotationAngle=smiData.RigidTransform(108).angle  RotationArbitraryAxis=smiData.RigidTransform(108).axis  FollAlignAxisA=+X  BaseAlignAxisA=+Y  FollAlignAxisB=+Y  BaseAlignAxisB=+Z  RotationSequenceAxes=FollowerAxes  RotationSequence=XYX  RotationSequenceAngles=[0 0 0]  RotationSequenceAnglesUnits=deg  RotationMatrix=[1 0 0; 0 1 0; 0 0 1]
  Transform81 : sm_lib/Frames and Transforms/Rigid Transform  TranslationMethod=Cartesian  TranslationStandardOffset=0  TranslationLengthUnit=mm  TranslationStandardAxis=+Z  TranslationCartesianOffset=smiData.RigidTransform(109).translation  TranslationROffset=0  TranslationROffsetUnits=m  TranslationZOffset=0  TranslationZOffsetUnits=m  TranslationThetaOffset=0  TranslationThetaOffsetUnits=deg  RotationMethod=ArbitraryAxis  RotationAngleUnits=rad  RotationStandardAxis=+Z  RotationAngle=smiData.RigidTransform(109).angle  RotationArbitraryAxis=smiData.RigidTransform(109).axis  FollAlignAxisA=+X  BaseAlignAxisA=+Y  FollAlignAxisB=+Y  BaseAlignAxisB=+Z  RotationSequenceAxes=FollowerAxes  RotationSequence=XYX  RotationSequenceAngles=[0 0 0]  RotationSequenceAnglesUnits=deg  RotationMatrix=[1 0 0; 0 1 0; 0 0 1]
  Transform82 : sm_lib/Frames and Transforms/Rigid Transform  TranslationMethod=Cartesian  TranslationStandardOffset=0  TranslationLengthUnit=mm  TranslationStandardAxis=+Z  TranslationCartesianOffset=smiData.RigidTransform(110).translation  TranslationROffset=0  TranslationROffsetUnits=m  TranslationZOffset=0  TranslationZOffsetUnits=m  TranslationThetaOffset=0  TranslationThetaOffsetUnits=deg  RotationMethod=ArbitraryAxis  RotationAngleUnits=rad  RotationStandardAxis=+Z  RotationAngle=smiData.RigidTransform(110).angle  RotationArbitraryAxis=smiData.RigidTransform(110).axis  FollAlignAxisA=+X  BaseAlignAxisA=+Y  FollAlignAxisB=+Y  BaseAlignAxisB=+Z  RotationSequenceAxes=FollowerAxes  RotationSequence=XYX  RotationSequenceAngles=[0 0 0]  RotationSequenceAnglesUnits=deg  RotationMatrix=[1 0 0; 0 1 0; 0 0 1]
  Transform83 : sm_lib/Frames and Transforms/Rigid Transform  TranslationMethod=Cartesian  TranslationStandardOffset=0  TranslationLengthUnit=mm  TranslationStandardAxis=+Z  TranslationCartesianOffset=smiData.RigidTransform(111).translation  TranslationROffset=0  TranslationROffsetUnits=m  TranslationZOffset=0  TranslationZOffsetUnits=m  TranslationThetaOffset=0  TranslationThetaOffsetUnits=deg  RotationMethod=ArbitraryAxis  RotationAngleUnits=rad  RotationStandardAxis=+Z  RotationAngle=smiData.RigidTransform(111).angle  RotationArbitraryAxis=smiData.RigidTransform(111).axis  FollAlignAxisA=+X  BaseAlignAxisA=+Y  FollAlignAxisB=+Y  BaseAlignAxisB=+Z  RotationSequenceAxes=FollowerAxes  RotationSequence=XYX  RotationSequenceAngles=[0 0 0]  RotationSequenceAnglesUnits=deg  RotationMatrix=[1 0 0; 0 1 0; 0 0 1]
  Transform84 : sm_lib/Frames and Transforms/Rigid Transform  TranslationMethod=Cartesian  TranslationStandardOffset=0  TranslationLengthUnit=mm  TranslationStandardAxis=+Z  TranslationCartesianOffset=smiData.RigidTransform(112).translation  TranslationROffset=0  TranslationROffsetUnits=m  TranslationZOffset=0  TranslationZOffsetUnits=m  TranslationThetaOffset=0  TranslationThetaOffsetUnits=deg  RotationMethod=ArbitraryAxis  RotationAngleUnits=rad  RotationStandardAxis=+Z  RotationAngle=smiData.RigidTransform(112).angle  RotationArbitraryAxis=smiData.RigidTransform(112).axis  FollAlignAxisA=+X  BaseAlignAxisA=+Y  FollAlignAxisB=+Y  BaseAlignAxisB=+Z  RotationSequenceAxes=FollowerAxes  RotationSequence=XYX  RotationSequenceAngles=[0 0 0]  RotationSequenceAnglesUnits=deg  RotationMatrix=[1 0 0; 0 1 0; 0 0 1]
  Transform85 : sm_lib/Frames and Transforms/Rigid Transform  TranslationMethod=Cartesian  TranslationStandardOffset=0  TranslationLengthUnit=mm  TranslationStandardAxis=+Z  TranslationCartesianOffset=smiData.RigidTransform(113).translation  TranslationROffset=0  TranslationROffsetUnits=m  TranslationZOffset=0  TranslationZOffsetUnits=m  TranslationThetaOffset=0  TranslationThetaOffsetUnits=deg  RotationMethod=ArbitraryAxis  RotationAngleUnits=rad  RotationStandardAxis=+Z  RotationAngle=smiData.RigidTransform(113).angle  RotationArbitraryAxis=smiData.RigidTransform(113).axis  FollAlignAxisA=+X  BaseAlignAxisA=+Y  FollAlignAxisB=+Y  BaseAlignAxisB=+Z  RotationSequenceAxes=FollowerAxes  RotationSequence=XYX  RotationSequenceAngles=[0 0 0]  RotationSequenceAnglesUnits=deg  RotationMatrix=[1 0 0; 0 1 0; 0 0 1]
  Transform86 : sm_lib/Frames and Transforms/Rigid Transform  TranslationMethod=Cartesian  TranslationStandardOffset=0  TranslationLengthUnit=mm  TranslationStandardAxis=+Z  TranslationCartesianOffset=smiData.RigidTransform(114).translation  TranslationROffset=0  TranslationROffsetUnits=m  TranslationZOffset=0  TranslationZOffsetUnits=m  TranslationThetaOffset=0  TranslationThetaOffsetUnits=deg  RotationMethod=ArbitraryAxis  RotationAngleUnits=rad  RotationStandardAxis=+Z  RotationAngle=smiData.RigidTransform(114).angle  RotationArbitraryAxis=smiData.RigidTransform(114).axis  FollAlignAxisA=+X  BaseAlignAxisA=+Y  FollAlignAxisB=+Y  BaseAlignAxisB=+Z  RotationSequenceAxes=FollowerAxes  RotationSequence=XYX  RotationSequenceAngles=[0 0 0]  RotationSequenceAnglesUnits=deg  RotationMatrix=[1 0 0; 0 1 0; 0 0 1]
  Transform87 : sm_lib/Frames and Transforms/Rigid Transform  TranslationMethod=Cartesian  TranslationStandardOffset=0  TranslationLengthUnit=mm  TranslationStandardAxis=+Z  TranslationCartesianOffset=smiData.RigidTransform(115).translation  TranslationROffset=0  TranslationROffsetUnits=m  TranslationZOffset=0  TranslationZOffsetUnits=m  TranslationThetaOffset=0  TranslationThetaOffsetUnits=deg  RotationMethod=ArbitraryAxis  RotationAngleUnits=rad  RotationStandardAxis=+Z  RotationAngle=smiData.RigidTransform(115).angle  RotationArbitraryAxis=smiData.RigidTransform(115).axis  FollAlignAxisA=+X  BaseAlignAxisA=+Y  FollAlignAxisB=+Y  BaseAlignAxisB=+Z  RotationSequenceAxes=FollowerAxes  RotationSequence=XYX  RotationSequenceAngles=[0 0 0]  RotationSequenceAnglesUnits=deg  RotationMatrix=[1 0 0; 0 1 0; 0 0 1]
  Transform88 : sm_lib/Frames and Transforms/Rigid Transform  TranslationMethod=Cartesian  TranslationStandardOffset=0  TranslationLengthUnit=mm  TranslationStandardAxis=+Z  TranslationCartesianOffset=smiData.RigidTransform(116).translation  TranslationROffset=0  TranslationROffsetUnits=m  TranslationZOffset=0  TranslationZOffsetUnits=m  TranslationThetaOffset=0  TranslationThetaOffsetUnits=deg  RotationMethod=ArbitraryAxis  RotationAngleUnits=rad  RotationStandardAxis=+Z  RotationAngle=smiData.RigidTransform(116).angle  RotationArbitraryAxis=smiData.RigidTransform(116).axis  FollAlignAxisA=+X  BaseAlignAxisA=+Y  FollAlignAxisB=+Y  BaseAlignAxisB=+Z  RotationSequenceAxes=FollowerAxes  RotationSequence=XYX  RotationSequenceAngles=[0 0 0]  RotationSequenceAnglesUnits=deg  RotationMatrix=[1 0 0; 0 1 0; 0 0 1]
  Transform89 : sm_lib/Frames and Transforms/Rigid Transform  TranslationMethod=Cartesian  TranslationStandardOffset=0  TranslationLengthUnit=mm  TranslationStandardAxis=+Z  TranslationCartesianOffset=smiData.RigidTransform(117).translation  TranslationROffset=0  TranslationROffsetUnits=m  TranslationZOffset=0  TranslationZOffsetUnits=m  TranslationThetaOffset=0  TranslationThetaOffsetUnits=deg  RotationMethod=ArbitraryAxis  RotationAngleUnits=rad  RotationStandardAxis=+Z  RotationAngle=smiData.RigidTransform(117).angle  RotationArbitraryAxis=smiData.RigidTransform(117).axis  FollAlignAxisA=+X  BaseAlignAxisA=+Y  FollAlignAxisB=+Y  BaseAlignAxisB=+Z  RotationSequenceAxes=FollowerAxes  RotationSequence=XYX  RotationSequenceAngles=[0 0 0]  RotationSequenceAnglesUnits=deg  RotationMatrix=[1 0 0; 0 1 0; 0 0 1]
  Transform9 : sm_lib/Frames and Transforms/Rigid Transform  TranslationMethod=Cartesian  TranslationStandardOffset=0  TranslationLengthUnit=mm  TranslationStandardAxis=+Z  TranslationCartesianOffset=smiData.RigidTransform(37).translation  TranslationROffset=0  TranslationROffsetUnits=m  TranslationZOffset=0  TranslationZOffsetUnits=m  TranslationThetaOffset=0  TranslationThetaOffsetUnits=deg  RotationMethod=ArbitraryAxis  RotationAngleUnits=rad  RotationStandardAxis=+Z  RotationAngle=smiData.RigidTransform(37).angle  RotationArbitraryAxis=smiData.RigidTransform(37).axis  FollAlignAxisA=+X  BaseAlignAxisA=+Y  FollAlignAxisB=+Y  BaseAlignAxisB=+Z  RotationSequenceAxes=FollowerAxes  RotationSequence=XYX  RotationSequenceAngles=[0 0 0]  RotationSequenceAnglesUnits=deg  RotationMatrix=[1 0 0; 0 1 0; 0 0 1]
  Transform90 : sm_lib/Frames and Transforms/Rigid Transform  TranslationMethod=Cartesian  TranslationStandardOffset=0  TranslationLengthUnit=mm  TranslationStandardAxis=+Z  TranslationCartesianOffset=smiData.RigidTransform(123).translation  TranslationROffset=0  TranslationROffsetUnits=m  TranslationZOffset=0  TranslationZOffsetUnits=m  TranslationThetaOffset=0  TranslationThetaOffsetUnits=deg  RotationMethod=ArbitraryAxis  RotationAngleUnits=rad  RotationStandardAxis=+Z  RotationAngle=smiData.RigidTransform(123).angle  RotationArbitraryAxis=smiData.RigidTransform(123).axis  FollAlignAxisA=+X  BaseAlignAxisA=+Y  FollAlignAxisB=+Y  BaseAlignAxisB=+Z  RotationSequenceAxes=FollowerAxes  RotationSequence=XYX  RotationSequenceAngles=[0 0 0]  RotationSequenceAnglesUnits=deg  RotationMatrix=[1 0 0; 0 1 0; 0 0 1]
  Transform91 : sm_lib/Frames and Transforms/Rigid Transform  TranslationMethod=Cartesian  TranslationStandardOffset=0  TranslationLengthUnit=mm  TranslationStandardAxis=+Z  TranslationCartesianOffset=smiData.RigidTransform(124).translation  TranslationROffset=0  TranslationROffsetUnits=m  TranslationZOffset=0  TranslationZOffsetUnits=m  TranslationThetaOffset=0  TranslationThetaOffsetUnits=deg  RotationMethod=ArbitraryAxis  RotationAngleUnits=rad  RotationStandardAxis=+Z  RotationAngle=smiData.RigidTransform(124).angle  RotationArbitraryAxis=smiData.RigidTransform(124).axis  FollAlignAxisA=+X  BaseAlignAxisA=+Y  FollAlignAxisB=+Y  BaseAlignAxisB=+Z  RotationSequenceAxes=FollowerAxes  RotationSequence=XYX  RotationSequenceAngles=[0 0 0]  RotationSequenceAnglesUnits=deg  RotationMatrix=[1 0 0; 0 1 0; 0 0 1]
  Transform92 : sm_lib/Frames and Transforms/Rigid Transform  TranslationMethod=Cartesian  TranslationStandardOffset=0  TranslationLengthUnit=mm  TranslationStandardAxis=+Z  TranslationCartesianOffset=smiData.RigidTransform(125).translation  TranslationROffset=0  TranslationROffsetUnits=m  TranslationZOffset=0  TranslationZOffsetUnits=m  TranslationThetaOffset=0  TranslationThetaOffsetUnits=deg  RotationMethod=ArbitraryAxis  RotationAngleUnits=rad  RotationStandardAxis=+Z  RotationAngle=smiData.RigidTransform(125).angle  RotationArbitraryAxis=smiData.RigidTransform(125).axis  FollAlignAxisA=+X  BaseAlignAxisA=+Y  FollAlignAxisB=+Y  BaseAlignAxisB=+Z  RotationSequenceAxes=FollowerAxes  RotationSequence=XYX  RotationSequenceAngles=[0 0 0]  RotationSequenceAnglesUnits=deg  RotationMatrix=[1 0 0; 0 1 0; 0 0 1]
  Transform93 : sm_lib/Frames and Transforms/Rigid Transform  TranslationMethod=Cartesian  TranslationStandardOffset=0  TranslationLengthUnit=mm  TranslationStandardAxis=+Z  TranslationCartesianOffset=smiData.RigidTransform(126).translation  TranslationROffset=0  TranslationROffsetUnits=m  TranslationZOffset=0  TranslationZOffsetUnits=m  TranslationThetaOffset=0  TranslationThetaOffsetUnits=deg  RotationMethod=ArbitraryAxis  RotationAngleUnits=rad  RotationStandardAxis=+Z  RotationAngle=smiData.RigidTransform(126).angle  RotationArbitraryAxis=smiData.RigidTransform(126).axis  FollAlignAxisA=+X  BaseAlignAxisA=+Y  FollAlignAxisB=+Y  BaseAlignAxisB=+Z  RotationSequenceAxes=FollowerAxes  RotationSequence=XYX  RotationSequenceAngles=[0 0 0]  RotationSequenceAnglesUnits=deg  RotationMatrix=[1 0 0; 0 1 0; 0 0 1]
  Transform94 : sm_lib/Frames and Transforms/Rigid Transform  TranslationMethod=Cartesian  TranslationStandardOffset=0  TranslationLengthUnit=mm  TranslationStandardAxis=+Z  TranslationCartesianOffset=smiData.RigidTransform(127).translation  TranslationROffset=0  TranslationROffsetUnits=m  TranslationZOffset=0  TranslationZOffsetUnits=m  TranslationThetaOffset=0  TranslationThetaOffsetUnits=deg  RotationMethod=ArbitraryAxis  RotationAngleUnits=rad  RotationStandardAxis=+Z  RotationAngle=smiData.RigidTransform(127).angle  RotationArbitraryAxis=smiData.RigidTransform(127).axis  FollAlignAxisA=+X  BaseAlignAxisA=+Y  FollAlignAxisB=+Y  BaseAlignAxisB=+Z  RotationSequenceAxes=FollowerAxes  RotationSequence=XYX  RotationSequenceAngles=[0 0 0]  RotationSequenceAnglesUnits=deg  RotationMatrix=[1 0 0; 0 1 0; 0 0 1]
  Transform95 : sm_lib/Frames and Transforms/Rigid Transform  TranslationMethod=Cartesian  TranslationStandardOffset=0  TranslationLengthUnit=mm  TranslationStandardAxis=+Z  TranslationCartesianOffset=smiData.RigidTransform(128).translation  TranslationROffset=0  TranslationROffsetUnits=m  TranslationZOffset=0  TranslationZOffsetUnits=m  TranslationThetaOffset=0  TranslationThetaOffsetUnits=deg  RotationMethod=ArbitraryAxis  RotationAngleUnits=rad  RotationStandardAxis=+Z  RotationAngle=smiData.RigidTransform(128).angle  RotationArbitraryAxis=smiData.RigidTransform(128).axis  FollAlignAxisA=+X  BaseAlignAxisA=+Y  FollAlignAxisB=+Y  BaseAlignAxisB=+Z  RotationSequenceAxes=FollowerAxes  RotationSequence=XYX  RotationSequenceAngles=[0 0 0]  RotationSequenceAnglesUnits=deg  RotationMatrix=[1 0 0; 0 1 0; 0 0 1]
  Transform96 : sm_lib/Frames and Transforms/Rigid Transform  TranslationMethod=Cartesian  TranslationStandardOffset=0  TranslationLengthUnit=mm  TranslationStandardAxis=+Z  TranslationCartesianOffset=smiData.RigidTransform(129).translation  TranslationROffset=0  TranslationROffsetUnits=m  TranslationZOffset=0  TranslationZOffsetUnits=m  TranslationThetaOffset=0  TranslationThetaOffsetUnits=deg  RotationMethod=ArbitraryAxis  RotationAngleUnits=rad  RotationStandardAxis=+Z  RotationAngle=smiData.RigidTransform(129).angle  RotationArbitraryAxis=smiData.RigidTransform(129).axis  FollAlignAxisA=+X  BaseAlignAxisA=+Y  FollAlignAxisB=+Y  BaseAlignAxisB=+Z  RotationSequenceAxes=FollowerAxes  RotationSequence=XYX  RotationSequenceAngles=[0 0 0]  RotationSequenceAnglesUnits=deg  RotationMatrix=[1 0 0; 0 1 0; 0 0 1]
  Transform97 : sm_lib/Frames and Transforms/Rigid Transform  TranslationMethod=Cartesian  TranslationStandardOffset=0  TranslationLengthUnit=mm  TranslationStandardAxis=+Z  TranslationCartesianOffset=smiData.RigidTransform(134).translation  TranslationROffset=0  TranslationROffsetUnits=m  TranslationZOffset=0  TranslationZOffsetUnits=m  TranslationThetaOffset=0  TranslationThetaOffsetUnits=deg  RotationMethod=ArbitraryAxis  RotationAngleUnits=rad  RotationStandardAxis=+Z  RotationAngle=smiData.RigidTransform(134).angle  RotationArbitraryAxis=smiData.RigidTransform(134).axis  FollAlignAxisA=+X  BaseAlignAxisA=+Y  FollAlignAxisB=+Y  BaseAlignAxisB=+Z  RotationSequenceAxes=FollowerAxes  RotationSequence=XYX  RotationSequenceAngles=[0 0 0]  RotationSequenceAnglesUnits=deg  RotationMatrix=[1 0 0; 0 1 0; 0 0 1]
  Transform98 : sm_lib/Frames and Transforms/Rigid Transform  TranslationMethod=Cartesian  TranslationStandardOffset=0  TranslationLengthUnit=mm  TranslationStandardAxis=+Z  TranslationCartesianOffset=smiData.RigidTransform(135).translation  TranslationROffset=0  TranslationROffsetUnits=m  TranslationZOffset=0  TranslationZOffsetUnits=m  TranslationThetaOffset=0  TranslationThetaOffsetUnits=deg  RotationMethod=ArbitraryAxis  RotationAngleUnits=rad  RotationStandardAxis=+Z  RotationAngle=smiData.RigidTransform(135).angle  RotationArbitraryAxis=smiData.RigidTransform(135).axis  FollAlignAxisA=+X  BaseAlignAxisA=+Y  FollAlignAxisB=+Y  BaseAlignAxisB=+Z  RotationSequenceAxes=FollowerAxes  RotationSequence=XYX  RotationSequenceAngles=[0 0 0]  RotationSequenceAnglesUnits=deg  RotationMatrix=[1 0 0; 0 1 0; 0 0 1]
  Transform99 : sm_lib/Frames and Transforms/Rigid Transform  TranslationMethod=Cartesian  TranslationStandardOffset=0  TranslationLengthUnit=mm  TranslationStandardAxis=+Z  TranslationCartesianOffset=smiData.RigidTransform(136).translation  TranslationROffset=0  TranslationROffsetUnits=m  TranslationZOffset=0  TranslationZOffsetUnits=m  TranslationThetaOffset=0  TranslationThetaOffsetUnits=deg  RotationMethod=ArbitraryAxis  RotationAngleUnits=rad  RotationStandardAxis=+Z  RotationAngle=smiData.RigidTransform(136).angle  RotationArbitraryAxis=smiData.RigidTransform(136).axis  FollAlignAxisA=+X  BaseAlignAxisA=+Y  FollAlignAxisB=+Y  BaseAlignAxisB=+Z  RotationSequenceAxes=FollowerAxes  RotationSequence=XYX  RotationSequenceAngles=[0 0 0]  RotationSequenceAnglesUnits=deg  RotationMatrix=[1 0 0; 0 1 0; 0 0 1]
  micro_usb_1_RIGID : Subsystem
  F : PMIOPort  Side=Left
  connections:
  Assembly2_1_RIGID/RConn1 -- Transform/LConn1 -- Transform1/LConn1 -- Transform10/LConn1 -- Transform100/LConn1 -- Transform101/LConn1 -- Transform102/LConn1 -- Transform103/LConn1 -- Transform104/LConn1 -- Transform105/LConn1 -- Transform106/LConn1 -- Transform107/LConn1 -- Transform108/LConn1 -- Transform109/LConn1 -- Transform11/LConn1 -- Transform110/LConn1 -- Transform111/LConn1 -- Transform112/LConn1 -- Transform113/LConn1 -- Transform12/LConn1 -- Transform13/LConn1 -- Transform14/LConn1 -- Transform15/LConn1 -- Transform16/LConn1 -- Transform17/LConn1 -- Transform18/LConn1 -- Transform19/LConn1 -- Transform2/LConn1 -- Transform20/LConn1 -- Transform21/LConn1 -- Transform22/LConn1 -- Transform23/LConn1 -- Transform24/LConn1 -- Transform25/LConn1 -- Transform26/LConn1 -- Transform27/LConn1 -- Transform28/LConn1 -- Transform29/LConn1 -- Transform3/LConn1 -- Transform30/LConn1 -- Transform31/LConn1 -- Transform32/LConn1 -- Transform33/LConn1 -- Transform34/LConn1 -- Transform35/LConn1 -- Transform36/LConn1 -- Transform37/LConn1 -- Transform38/LConn1 -- Transform39/LConn1 -- Transform4/LConn1 -- Transform40/LConn1 -- Transform41/LConn1 -- Transform42/LConn1 -- Transform43/LConn1 -- Transform44/LConn1 -- Transform45/LConn1 -- Transform98/LConn1 -- Transform99/LConn1 -- Transform97/LConn1 -- Transform96/LConn1 -- Transform95/LConn1 -- Transform94/LConn1 -- Transform93/LConn1 -- Transform92/LConn1 -- Transform91/LConn1 -- Transform90/LConn1 -- Transform9/LConn1 -- Transform89/LConn1 -- Transform88/LConn1 -- Transform87/LConn1 -- Transform86/LConn1 -- Transform85/LConn1 -- Transform84/LConn1 -- Transform83/LConn1 -- Transform82/LConn1 -- Transform81/LConn1 -- Transform80/LConn1 -- Transform8/LConn1 -- Transform79/LConn1 -- Transform78/LConn1 -- Transform77/LConn1 -- Transform76/LConn1 -- Transform75/LConn1 -- Transform74/LConn1 -- Transform73/LConn1 -- Transform72/LConn1 -- Transform71/LConn1 -- Transform70/LConn1 -- Transform7/LConn1 -- Transform69/LConn1 -- Transform68/LConn1 -- Transform67/LConn1 -- Transform66/LConn1 -- Transform65/LConn1 -- Transform64/LConn1 -- Transform63/LConn1 -- Transform62/LConn1 -- Transform61/LConn1 -- Transform60/LConn1 -- Transform6/LConn1 -- Transform59/LConn1 -- Transform58/LConn1 -- Transform57/LConn1 -- Transform56/LConn1 -- Transform55/LConn1 -- Transform54/LConn1 -- Transform53/LConn1 -- Transform52/LConn1 -- Transform51/LConn1 -- Transform50/LConn1 -- Transform5/LConn1 -- Transform49/LConn1 -- Transform48/LConn1 -- Transform47/LConn1 -- Transform46/LConn1 -- Button_assembly_microbit_3_RIGID/RConn1 -- ReferenceFrame/RConn1 -- Button_assembly_microbit_2_RIGID/RConn1 -- Button_assembly_microbit_1_RIGID/RConn1
  Transform/RConn1 -- F/RConn1
  Resistance_1_RIGID/LConn1 -- Transform9/RConn1
  Carte_microbit_1_RIGID/LConn1 -- Transform99/RConn1
  Resistance_41_RIGID/LConn1 -- Transform100/RConn1
  Resistance_42_RIGID/LConn1 -- Transform101/RConn1
  LED_18_RIGID/LConn1 -- Transform102/RConn1
  LED_19_RIGID/LConn1 -- Transform103/RConn1
  Pins_1_RIGID/LConn1 -- Transform104/RConn1
  LED_20_RIGID/LConn1 -- Transform105/RConn1
  Resistance_38_RIGID/LConn1 -- Transform106/RConn1
  LED_24_RIGID/LConn1 -- Transform107/RConn1
  LED_23_RIGID/LConn1 -- Transform108/RConn1
  Resistance_2_RIGID/LConn1 -- Transform10/RConn1
  Resistance_37_RIGID/LConn1 -- Transform109/RConn1
  Pins_2_RIGID/LConn1 -- Transform110/RConn1
  LED_25_RIGID/LConn1 -- Transform111/RConn1
  Resistance_45_RIGID/LConn1 -- Transform112/RConn1
  LED_21_RIGID/LConn1 -- Transform113/RConn1
  Resistance_9_RIGID/LConn1 -- Transform11/RConn1
  Resistance_13_RIGID/LConn1 -- Transform12/RConn1
  Resistance_14_RIGID/LConn1 -- Transform13/RConn1
  Resistance_16_RIGID/LConn1 -- Transform14/RConn1
  Resistance_17_RIGID/LConn1 -- Transform15/RConn1
  Resistance_3_RIGID/LConn1 -- Transform16/RConn1
  Resistance_11_RIGID/LConn1 -- Transform17/RConn1
  Resistance_4_RIGID/LConn1 -- Transform18/RConn1
  Resistance_6_RIGID/LConn1 -- Transform1/RConn1
  Resistance_7_RIGID/LConn1 -- Transform19/RConn1
  Resistance_18_RIGID/LConn1 -- Transform20/RConn1
  Resistance_19_RIGID/LConn1 -- Transform21/RConn1
  Resistance_15_RIGID/LConn1 -- Transform22/RConn1
  Resistance_21_RIGID/LConn1 -- Transform23/RConn1
  Resistance_23_RIGID/LConn1 -- Transform24/RConn1
  Condensateur_cylindrique_9_RIGID/LConn1 -- Transform25/RConn1
  Condensateur_6_RIGID/LConn1 -- Transform26/RConn1
  LED_1_RIGID/LConn1 -- Transform27/RConn1
  Condensateur_cylindrique_2_RIGID/LConn1 -- Transform28/RConn1
  Resistance_10_RIGID/LConn1 -- Transform2/RConn1
  LED_3_RIGID/LConn1 -- Transform29/RConn1
  LED_2_RIGID/LConn1 -- Transform30/RConn1
  LED_4_RIGID/LConn1 -- Transform31/RConn1
  Condensateur_cylindrique_8_RIGID/LConn1 -- Transform32/RConn1
  Condensateur_2_RIGID/LConn1 -- Transform33/RConn1
  Resistance_25_RIGID/LConn1 -- Transform34/RConn1
  Condensateur_cylindrique_4_RIGID/LConn1 -- Transform35/RConn1
  Condensateur_cylindrique_5_RIGID/LConn1 -- Transform36/RConn1
  Condensateur_cylindrique_6_RIGID/LConn1 -- Transform37/RConn1
  Condensateur_cylindrique_7_RIGID/LConn1 -- Transform38/RConn1
  Resistance_5_RIGID/LConn1 -- Transform3/RConn1
  Condensateur_cylindrique_3_RIGID/LConn1 -- Transform39/RConn1
  Condensateur_3_RIGID/LConn1 -- Transform40/RConn1
  Condensateur_1_RIGID/LConn1 -- Transform41/RConn1
  Condensateur_4_RIGID/LConn1 -- Transform42/RConn1
  Condensateur_5_RIGID/LConn1 -- Transform43/RConn1
  Condensateur_cylindrique_1_RIGID/LConn1 -- Transform44/RConn1
  LED_8_RIGID/LConn1 -- Transform45/RConn1
  LED_11_RIGID/LConn1 -- Transform46/RConn1
  LED_6_RIGID/LConn1 -- Transform47/RConn1
  Circuit_integre_1_1_RIGID/LConn1 -- Transform48/RConn1
  Resistance_20_RIGID/LConn1 -- Transform4/RConn1
  LED_9_RIGID/LConn1 -- Transform49/RConn1
  LED_17_RIGID/LConn1 -- Transform50/RConn1
  LED_10_RIGID/LConn1 -- Transform51/RConn1
  Condensateur_cylindrique_16_RIGID/LConn1 -- Transform52/RConn1
  Circuit_integre_4_1_RIGID/LConn1 -- Transform53/RConn1
  Condensateur_cylindrique_19_RIGID/LConn1 -- Transform54/RConn1
  Circuit_integre_2_1_RIGID/LConn1 -- Transform55/RConn1
  Circuit_integre_5_1_RIGID/LConn1 -- Transform56/RConn1
  LED_7_RIGID/LConn1 -- Transform57/RConn1
  Condensateur_cylindrique_11_RIGID/LConn1 -- Transform58/RConn1
  Resistance_22_RIGID/LConn1 -- Transform5/RConn1
  Condensateur_cylindrique_10_RIGID/LConn1 -- Transform59/RConn1
  LED_14_RIGID/LConn1 -- Transform60/RConn1
  Texte_face_devant_1_RIGID/LConn1 -- Transform61/RConn1
  Connecteur_alimentation_1_RIGID/LConn1 -- Transform62/RConn1
  Condensateur_cylindrique_13_RIGID/LConn1 -- Transform63/RConn1
  Condensateur_cylindrique_15_RIGID/LConn1 -- Transform64/RConn1
  LED_5_RIGID/LConn1 -- Transform65/RConn1
  LED_15_RIGID/LConn1 -- Transform66/RConn1
  LED_12_RIGID/LConn1 -- Transform67/RConn1
  LED_16_RIGID/LConn1 -- Transform68/RConn1
  Resistance_24_RIGID/LConn1 -- Transform6/RConn1
  LED_13_RIGID/LConn1 -- Transform69/RConn1
  Circuit_integre_4_2_RIGID/LConn1 -- Transform70/RConn1
  Condensateur_cylindrique_12_RIGID/LConn1 -- Transform71/RConn1
  Circuit_integre_3_2_RIGID/LConn1 -- Transform72/RConn1
  Transform73/RConn1 -- micro_usb_1_RIGID/LConn1
  Circuit_integre_3_1_RIGID/LConn1 -- Transform74/RConn1
  Condensateur_cylindrique_14_RIGID/LConn1 -- Transform75/RConn1
  Condensateur_cylindrique_17_RIGID/LConn1 -- Transform76/RConn1
  Condensateur_cylindrique_18_RIGID/LConn1 -- Transform77/RConn1
  Resistance_30_RIGID/LConn1 -- Transform78/RConn1
  Resistance_12_RIGID/LConn1 -- Transform7/RConn1
  Resistance_32_RIGID/LConn1 -- Transform79/RConn1
  Condensateur_cylindrique_20_RIGID/LConn1 -- Transform80/RConn1
  Resistance_28_RIGID/LConn1 -- Transform81/RConn1
  Resistance_33_RIGID/LConn1 -- Transform82/RConn1
  Texte_derriere_1_RIGID/LConn1 -- Transform83/RConn1
  Resistance_29_RIGID/LConn1 -- Transform84/RConn1
  Resistance_34_RIGID/LConn1 -- Transform85/RConn1
  Resistance_27_RIGID/LConn1 -- Transform86/RConn1
  Lignes_face_arrire_1_RIGID/LConn1 -- Transform87/RConn1
  Antenne_1_RIGID/LConn1 -- Transform88/RConn1
  Resistance_8_RIGID/LConn1 -- Transform8/RConn1
  Slot_condensateur_1_RIGID/LConn1 -- Transform89/RConn1
  Resistance_35_RIGID/LConn1 -- Transform90/RConn1
  Resistance_36_RIGID/LConn1 -- Transform91/RConn1
  Resistance_26_RIGID/LConn1 -- Transform92/RConn1
  Resistance_31_RIGID/LConn1 -- Transform93/RConn1
  Resistance_44_RIGID/LConn1 -- Transform94/RConn1
  Resistance_39_RIGID/LConn1 -- Transform95/RConn1
  LED_22_RIGID/LConn1 -- Transform96/RConn1
  Resistance_40_RIGID/LConn1 -- Transform97/RConn1
  Resistance_43_RIGID/LConn1 -- Transform98/RConn1
